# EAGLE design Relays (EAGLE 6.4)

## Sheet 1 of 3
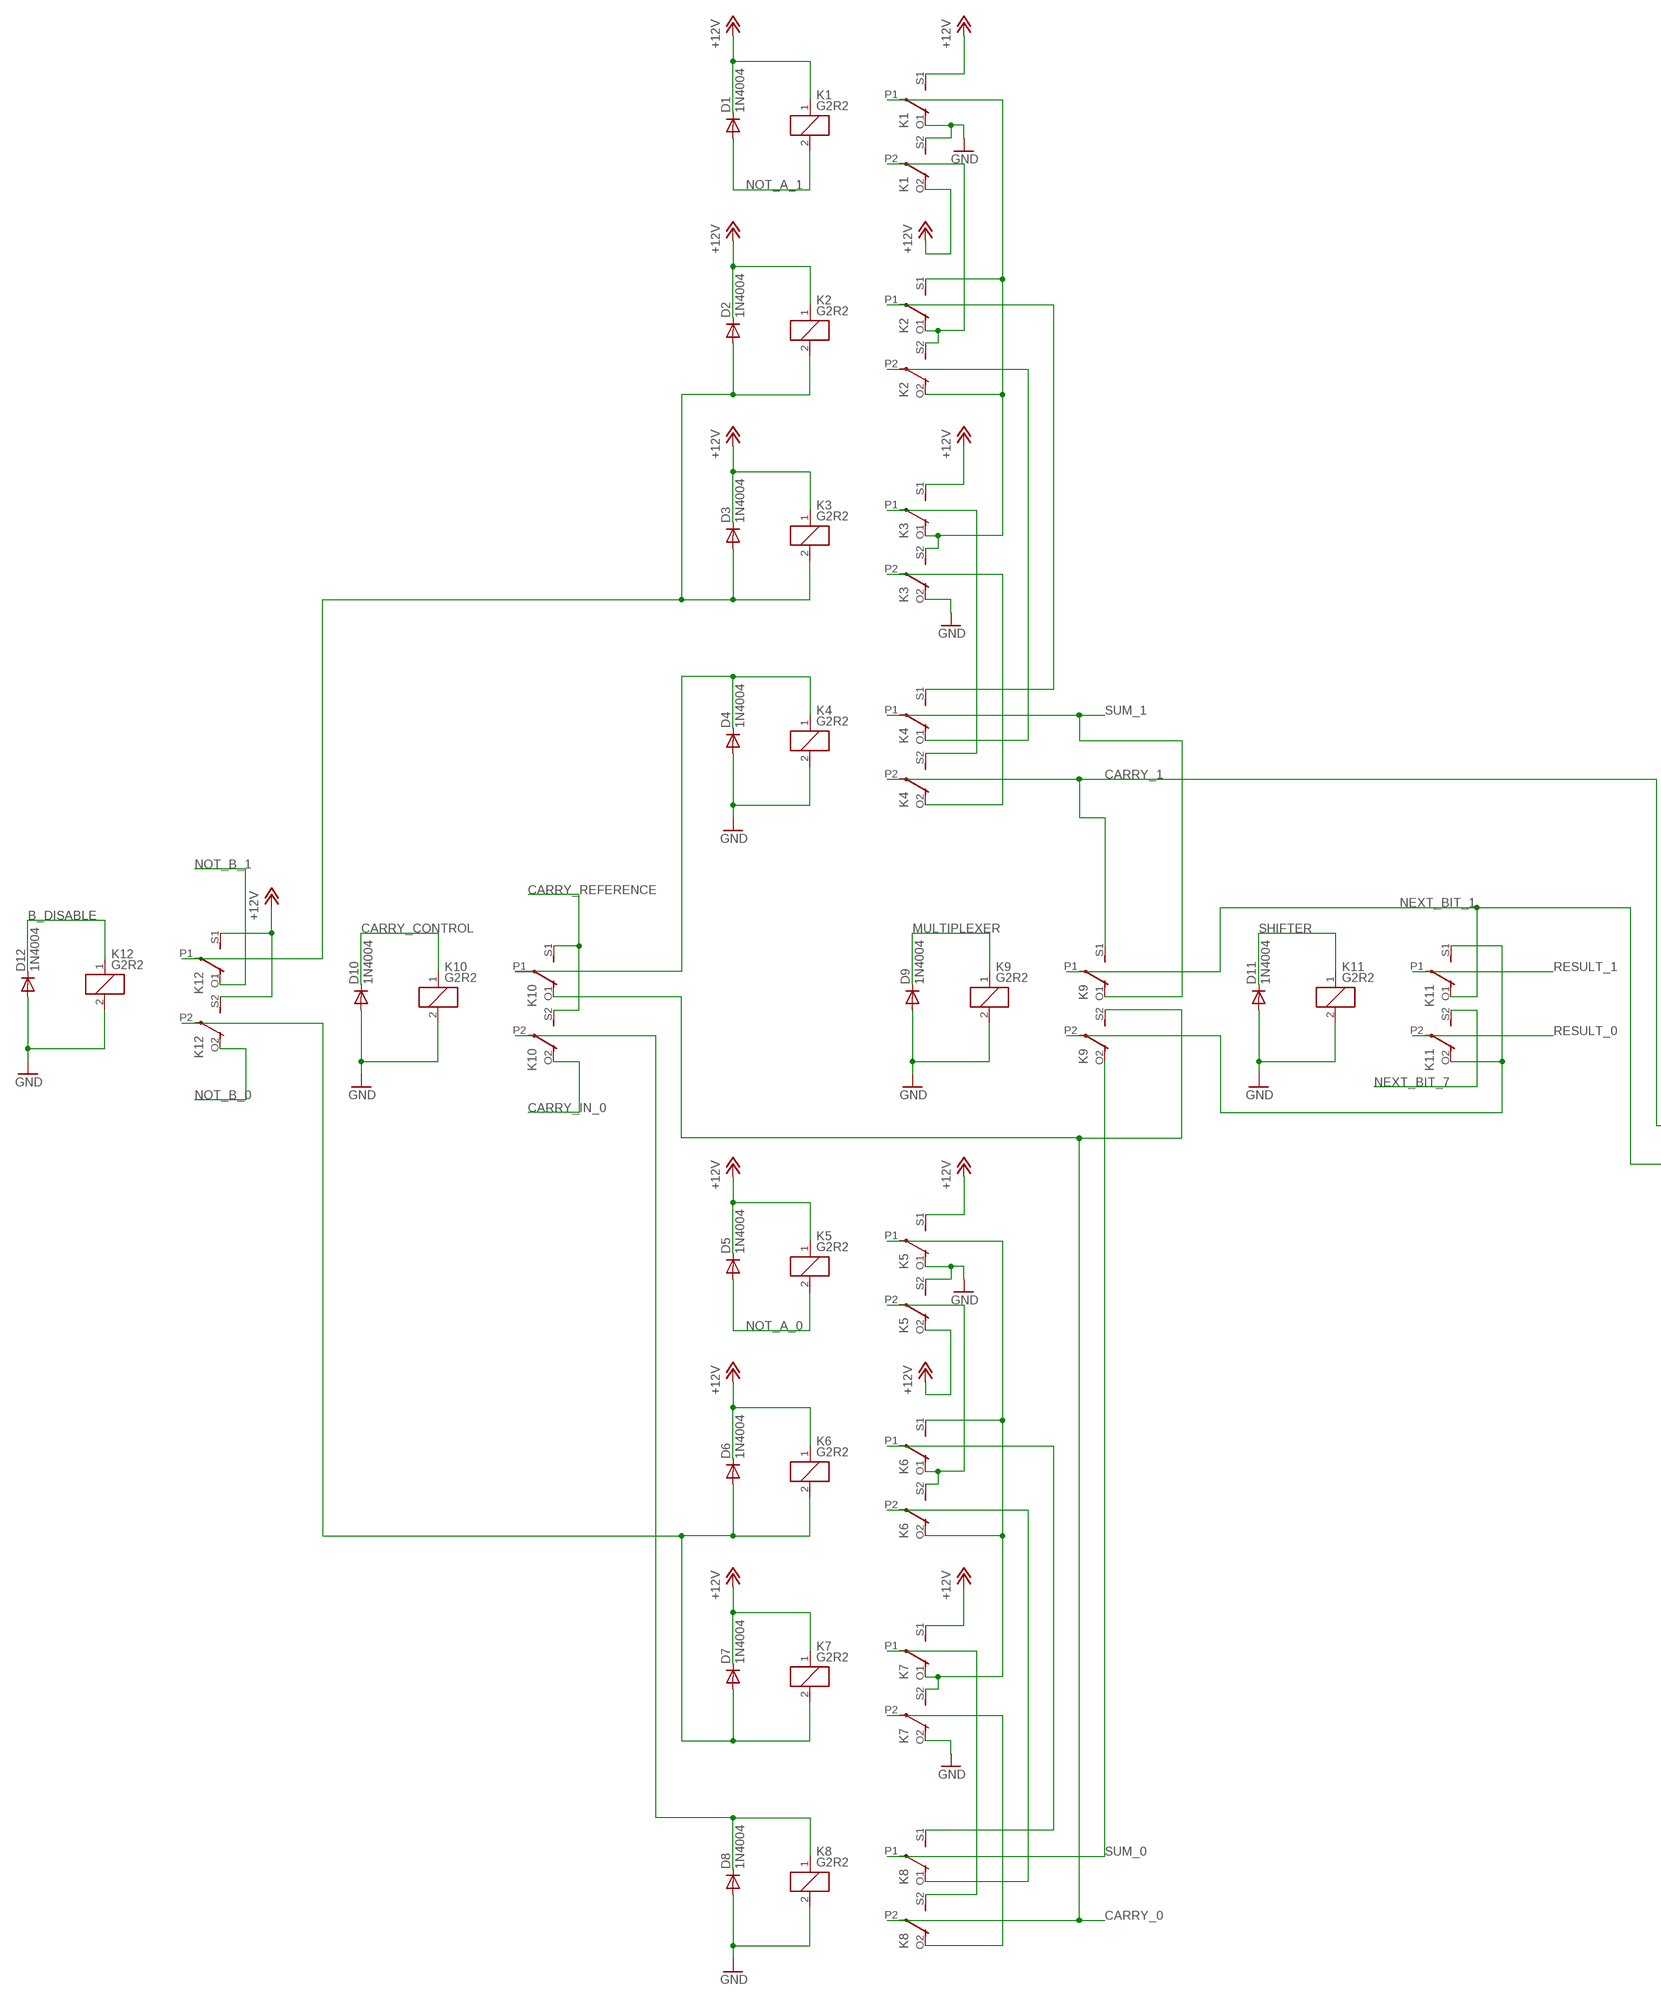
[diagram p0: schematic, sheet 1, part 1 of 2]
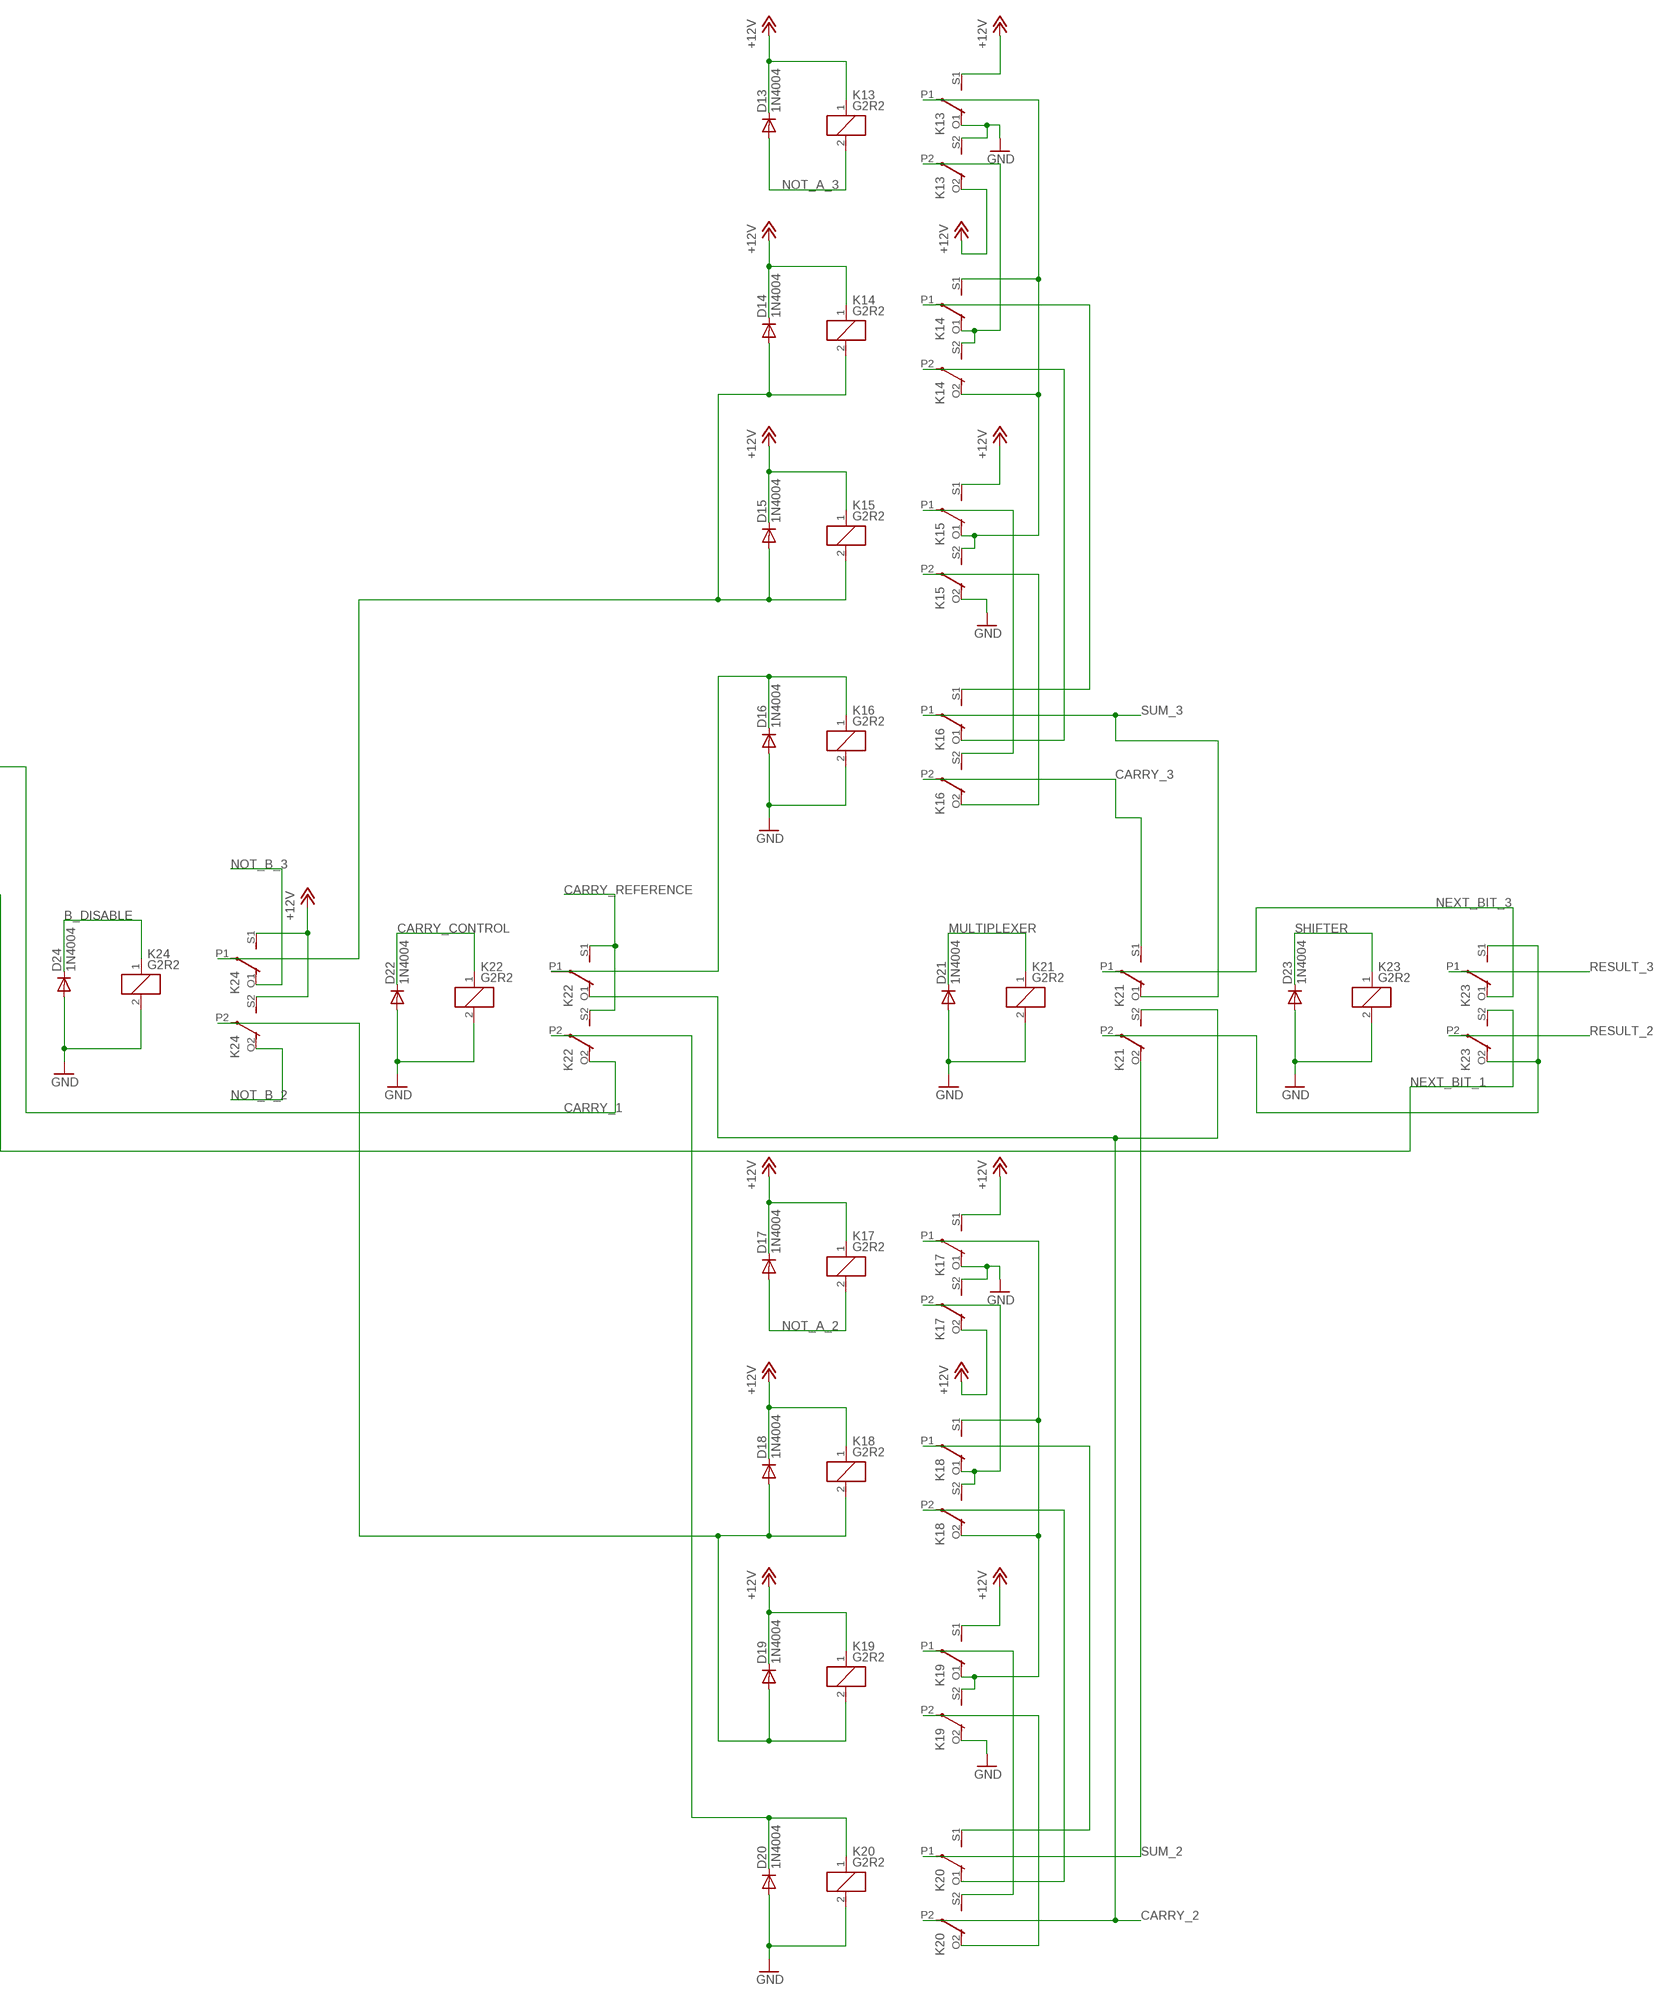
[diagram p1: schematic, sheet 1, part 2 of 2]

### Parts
D1  1N4004  [DO41-10]
D2  1N4004  [DO41-10]
D3  1N4004  [DO41-10]
D4  1N4004  [DO41-10]
D5  1N4004  [DO41-10]
D6  1N4004  [DO41-10]
D7  1N4004  [DO41-10]
D8  1N4004  [DO41-10]
D9  1N4004  [DO41-10]
D10  1N4004  [DO41-10]
D11  1N4004  [DO41-10]
D12  1N4004  [DO41-10]
D13  1N4004  [DO41-10]
D14  1N4004  [DO41-10]
D15  1N4004  [DO41-10]
D16  1N4004  [DO41-10]
D17  1N4004  [DO41-10]
D18  1N4004  [DO41-10]
D19  1N4004  [DO41-10]
D20  1N4004  [DO41-10]
D21  1N4004  [DO41-10]
D22  1N4004  [DO41-10]
D23  1N4004  [DO41-10]
D24  1N4004  [DO41-10]
K1  G2R2  [G2R2]
K2  G2R2  [G2R2]
K3  G2R2  [G2R2]
K4  G2R2  [G2R2]
K5  G2R2  [G2R2]
K6  G2R2  [G2R2]
K7  G2R2  [G2R2]
K8  G2R2  [G2R2]
K9  G2R2  [G2R2]
K10  G2R2  [G2R2]
K11  G2R2  [G2R2]
K12  G2R2  [G2R2]
K13  G2R2  [G2R2]
K14  G2R2  [G2R2]
K15  G2R2  [G2R2]
K16  G2R2  [G2R2]
K17  G2R2  [G2R2]
K18  G2R2  [G2R2]
K19  G2R2  [G2R2]
K20  G2R2  [G2R2]
K21  G2R2  [G2R2]
K22  G2R2  [G2R2]
K23  G2R2  [G2R2]
K24  G2R2  [G2R2]

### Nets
+12V [12V_Power]: D1.C D2.C D3.C D5.C D6.C D7.C D13.C D14.C D15.C D17.C D18.C D19.C K1.1 K1.O2(3:O) K1.S1(2:S) K2.1 K3.1 K3.S1(2:S) K5.1 K5.O2(3:O) K5.S1(2:S) K6.1 K7.1 K7.S1(2:S) K12.S1(2:S) K12.S2(3:S) K13.1 K13.O2(3:O) K13.S1(2:S) K14.1 K15.1 K15.S1(2:S) K17.1 K17.O2(3:O) K17.S1(2:S) K18.1 K19.1 K19.S1(2:S) K24.S1(2:S) K24.S2(3:S) ; also sheet 2,3
B_DISABLE [Relay_Interconnects]: D12.C D24.C K12.1 K24.1 ; also sheet 2,3
CARRY_0 [Relay_Interconnects]: K8.P2(3:P) K9.S2(3:S) K10.O1(2:O)
CARRY_1 [Relay_Interconnects]: K4.P2(3:P) K9.S1(2:S) K22.O2(3:O)
CARRY_2 [Relay_Interconnects]: K20.P2(3:P) K21.S2(3:S) K22.O1(2:O)
CARRY_3: K16.P2(3:P) K21.S1(2:S) ; also sheet 3
CARRY_CONTROL [Relay_Interconnects]: D10.C D22.C K10.1 K22.1 ; also sheet 2,3
CARRY_IN_0 [Relay_Interconnects]: K10.O2(3:O) ; also sheet 2
CARRY_REFERENCE [Relay_Interconnects]: K10.S1(2:S) K10.S2(3:S) K22.S1(2:S) K22.S2(3:S) ; also sheet 2,3
GND [Ground]: D4.A D8.A D9.A D10.A D11.A D12.A D16.A D20.A D21.A D22.A D23.A D24.A K1.O1(2:O) K1.S2(3:S) K3.O2(3:O) K4.2 K5.O1(2:O) K5.S2(3:S) K7.O2(3:O) K8.2 K9.2 K10.2 K11.2 K12.2 K13.O1(2:O) K13.S2(3:S) K15.O2(3:O) K16.2 K17.O1(2:O) K17.S2(3:S) K19.O2(3:O) K20.2 K21.2 K22.2 K23.2 K24.2 ; also sheet 2,3
MULTIPLEXER [Relay_Interconnects]: D9.C D21.C K9.1 K21.1 ; also sheet 2,3
N$1 [Relay_Interconnects]: D2.A D3.A K2.2 K3.2 K12.P1(2:P)
N$3 [Relay_Interconnects]: K9.P2(3:P) K11.O2(3:O) K11.S1(2:S)
N$5 [Relay_Interconnects]: D16.C K16.1 K22.P1(2:P)
N$6: K13.P2(3:P) K14.O1(2:O) K14.S2(3:S)
N$7 [Relay_Interconnects]: D4.C K4.1 K10.P1(2:P)
N$8 [Relay_Interconnects]: D8.C K8.1 K10.P2(3:P)
N$9: K2.P1(2:P) K4.S1(2:S)
N$10: K1.P2(3:P) K2.O1(2:O) K2.S2(3:S)
N$11: K5.P2(3:P) K6.O1(2:O) K6.S2(3:S)
N$12: K1.P1(2:P) K2.O2(3:O) K2.S1(2:S) K3.O1(2:O) K3.S2(3:S)
N$13: K5.P1(2:P) K6.O2(3:O) K6.S1(2:S) K7.O1(2:O) K7.S2(3:S)
N$14: K7.P2(3:P) K8.O2(3:O)
N$15: K3.P2(3:P) K4.O2(3:O)
N$16: K3.P1(2:P) K4.S2(3:S)
N$17: K2.P2(3:P) K4.O1(2:O)
N$18: K7.P1(2:P) K8.S2(3:S)
N$19: K6.P2(3:P) K8.O1(2:O)
N$20: K6.P1(2:P) K8.S1(2:S)
N$21: K13.P1(2:P) K14.O2(3:O) K14.S1(2:S) K15.O1(2:O) K15.S2(3:S)
N$22 [Relay_Interconnects]: D6.A D7.A K6.2 K7.2 K12.P2(3:P)
N$23: K15.P2(3:P) K16.O2(3:O)
N$24: K15.P1(2:P) K16.S2(3:S)
N$25: K14.P2(3:P) K16.O1(2:O)
N$26: K14.P1(2:P) K16.S1(2:S)
N$27 [Relay_Interconnects]: D20.C K20.1 K22.P2(3:P)
N$28: K17.P2(3:P) K18.O1(2:O) K18.S2(3:S)
N$29: K17.P1(2:P) K18.O2(3:O) K18.S1(2:S) K19.O1(2:O) K19.S2(3:S)
N$30: K19.P2(3:P) K20.O2(3:O)
N$31: K19.P1(2:P) K20.S2(3:S)
N$32: K18.P2(3:P) K20.O1(2:O)
N$33: K18.P1(2:P) K20.S1(2:S)
N$34 [Relay_Interconnects]: D14.A D15.A K14.2 K15.2 K24.P1(2:P)
N$35 [Relay_Interconnects]: D18.A D19.A K18.2 K19.2 K24.P2(3:P)
N$36 [Relay_Interconnects]: K21.P2(3:P) K23.O2(3:O) K23.S1(2:S)
NEXT_BIT_1 [Relay_Interconnects]: K9.P1(2:P) K11.O1(2:O) K23.S2(3:S)
NEXT_BIT_3 [Relay_Interconnects]: K21.P1(2:P) K23.O1(2:O) ; also sheet 3
NEXT_BIT_7 [Relay_Interconnects]: K11.S2(3:S) ; also sheet 3
NOT_A_0 [Relay_Interconnects]: D5.A K5.2 ; also sheet 3
NOT_A_1 [Relay_Interconnects]: D1.A K1.2 ; also sheet 3
NOT_A_2 [Relay_Interconnects]: D17.A K17.2 ; also sheet 3
NOT_A_3 [Relay_Interconnects]: D13.A K13.2 ; also sheet 3
NOT_B_0 [Relay_Interconnects]: K12.O2(3:O) ; also sheet 3
NOT_B_1 [Relay_Interconnects]: K12.O1(2:O) ; also sheet 3
NOT_B_2 [Relay_Interconnects]: K24.O2(3:O) ; also sheet 3
NOT_B_3 [Relay_Interconnects]: K24.O1(2:O) ; also sheet 3
RESULT_0 [Relay_Interconnects]: K11.P2(3:P) ; also sheet 3
RESULT_1 [Relay_Interconnects]: K11.P1(2:P) ; also sheet 3
RESULT_2 [Relay_Interconnects]: K23.P2(3:P) ; also sheet 3
RESULT_3 [Relay_Interconnects]: K23.P1(2:P) ; also sheet 3
SHIFTER [Relay_Interconnects]: D11.C D23.C K11.1 K23.1 ; also sheet 2,3
SUM_0: K8.P1(2:P) K9.O2(3:O)
SUM_1 [Relay_Interconnects]: K4.P1(2:P) K9.O1(2:O)
SUM_2: K20.P1(2:P) K21.O2(3:O)
SUM_3 [Relay_Interconnects]: K16.P1(2:P) K21.O1(2:O)

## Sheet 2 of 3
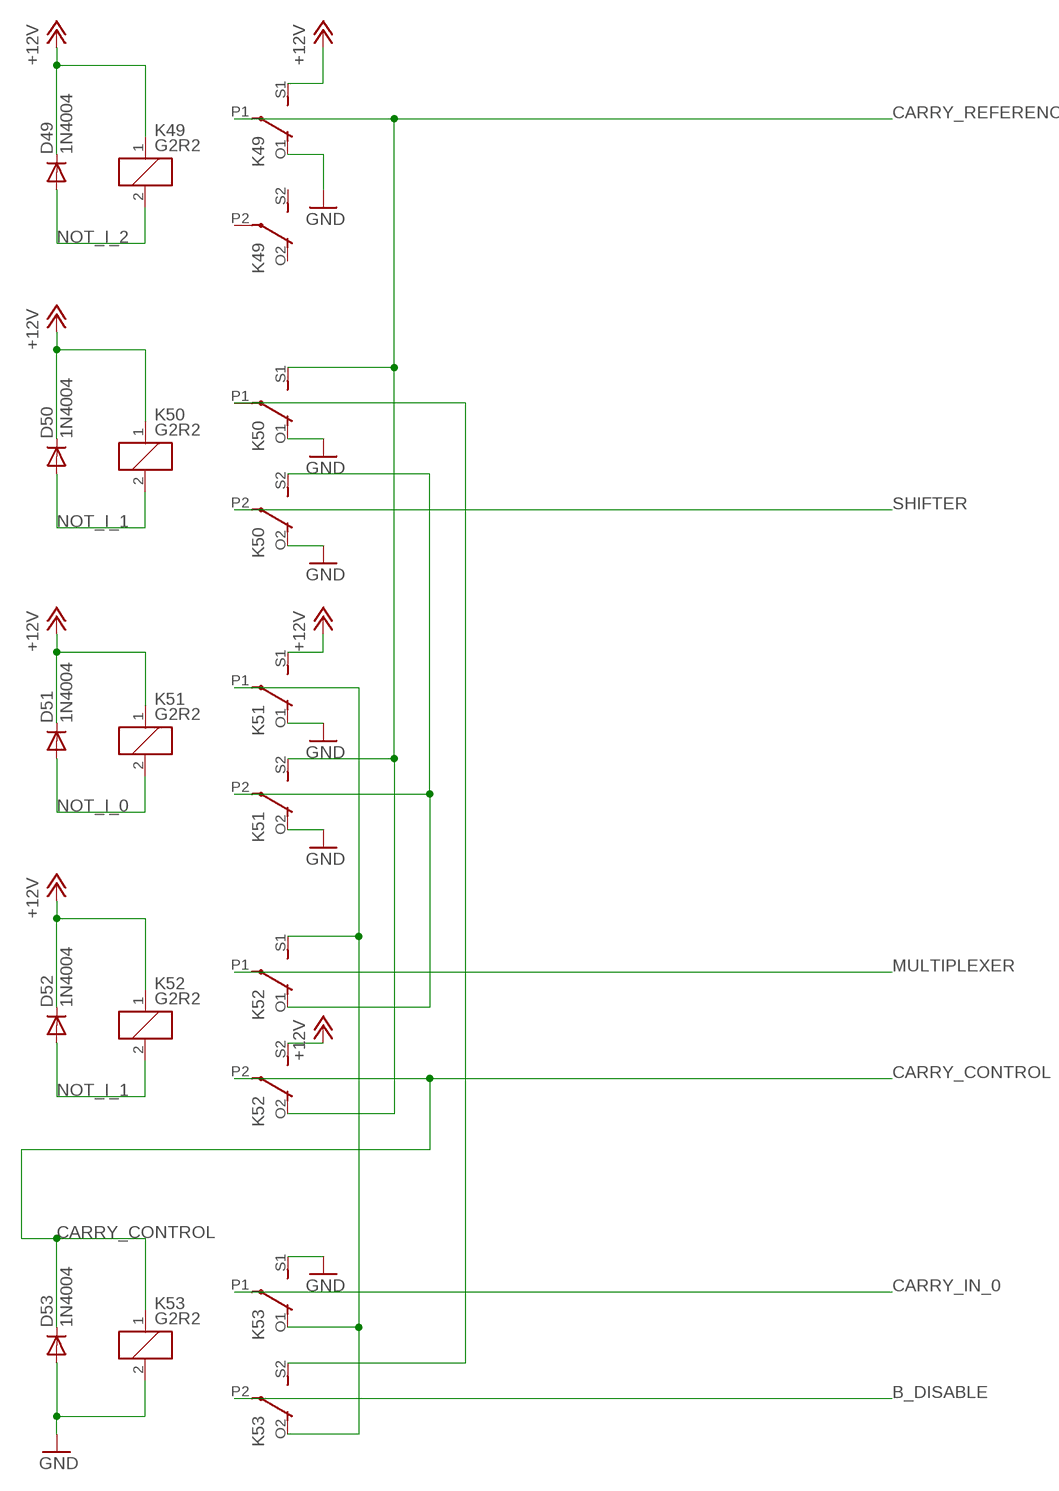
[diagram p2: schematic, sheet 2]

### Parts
D49  1N4004  [DO41-10]
D50  1N4004  [DO41-10]
D51  1N4004  [DO41-10]
D52  1N4004  [DO41-10]
D53  1N4004  [DO41-10]
K49  G2R2  [G2R2]
K50  G2R2  [G2R2]
K51  G2R2  [G2R2]
K52  G2R2  [G2R2]
K53  G2R2  [G2R2]

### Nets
+12V [12V_Power]: D49.C D50.C D51.C D52.C K49.1 K49.S1(2:S) K50.1 K51.1 K51.S1(2:S) K52.1 K52.S2(3:S) ; also sheet 1,3
B_DISABLE [Relay_Interconnects]: K53.P2(3:P) ; also sheet 1,3
CARRY_CONTROL [Relay_Interconnects]: D53.C K52.P2(3:P) K53.1 ; also sheet 1,3
CARRY_IN_0 [Relay_Interconnects]: K53.P1(2:P) ; also sheet 1
CARRY_REFERENCE [Relay_Interconnects]: K49.P1(2:P) K50.S1(2:S) K51.S2(3:S) K52.O2(3:O) ; also sheet 1,3
GND [Ground]: D53.A K49.O1(2:O) K50.O1(2:O) K50.O2(3:O) K51.O1(2:O) K51.O2(3:O) K53.2 K53.S1(2:S) ; also sheet 1,3
MULTIPLEXER [Relay_Interconnects]: K52.P1(2:P) ; also sheet 1,3
N$4: K50.S2(3:S) K51.P2(3:P) K52.O1(2:O)
N$71: K50.P1(2:P) K53.S2(3:S)
N$72: K51.P1(2:P) K52.S1(2:S) K53.O1(2:O) K53.O2(3:O)
NOT_I_0: D51.A K51.2 ; also sheet 3
NOT_I_1: D50.A D52.A K50.2 K52.2 ; also sheet 3
NOT_I_2: D49.A K49.2 ; also sheet 3
SHIFTER [Relay_Interconnects]: K50.P2(3:P) ; also sheet 1,3
Unconnected: K49.O2(3:O) K49.P2(3:P) K49.S2(3:S)

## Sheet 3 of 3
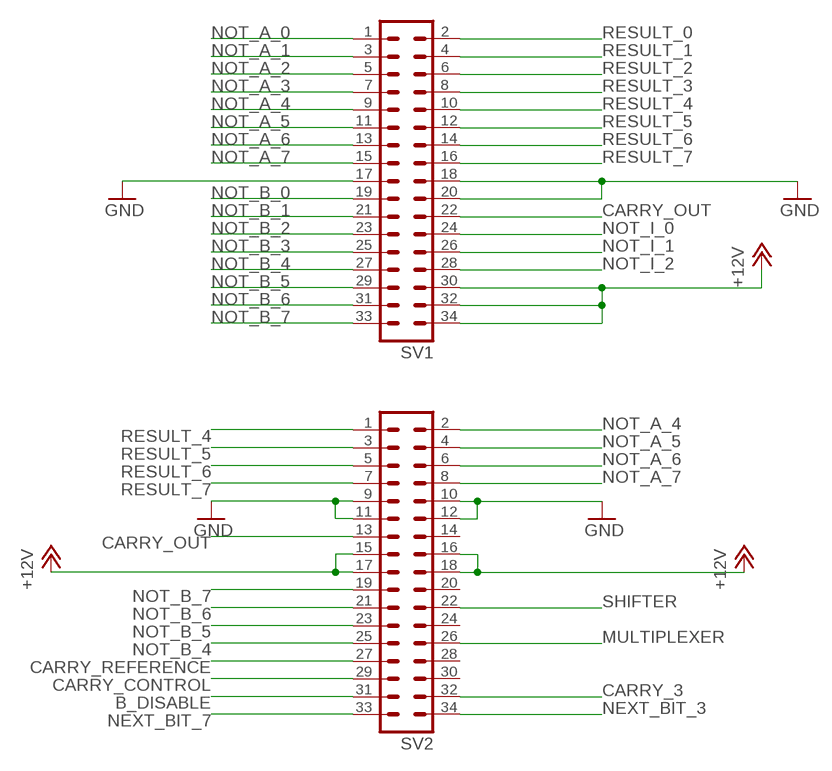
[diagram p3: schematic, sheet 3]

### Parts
SV1  ML34  [ML34]
SV2  ML34  [ML34]

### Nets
+12V [12V_Power]: SV1.30 SV1.32 SV1.34 SV2.15 SV2.16 SV2.17 SV2.18 ; also sheet 1,2
B_DISABLE [Relay_Interconnects]: SV2.31 ; also sheet 1,2
CARRY_3: SV2.32 ; also sheet 1
CARRY_CONTROL [Relay_Interconnects]: SV2.29 ; also sheet 1,2
CARRY_OUT [Relay_Interconnects]: SV1.22 SV2.13
CARRY_REFERENCE [Relay_Interconnects]: SV2.27 ; also sheet 1,2
GND [Ground]: SV1.17 SV1.18 SV1.20 SV2.9 SV2.10 SV2.11 SV2.12 ; also sheet 1,2
MULTIPLEXER [Relay_Interconnects]: SV2.26 ; also sheet 1,2
NEXT_BIT_3 [Relay_Interconnects]: SV2.34 ; also sheet 1
NEXT_BIT_7 [Relay_Interconnects]: SV2.33 ; also sheet 1
NOT_A_0 [Relay_Interconnects]: SV1.1 ; also sheet 1
NOT_A_1 [Relay_Interconnects]: SV1.3 ; also sheet 1
NOT_A_2 [Relay_Interconnects]: SV1.5 ; also sheet 1
NOT_A_3 [Relay_Interconnects]: SV1.7 ; also sheet 1
NOT_A_4 [Relay_Interconnects]: SV1.9 SV2.2
NOT_A_5 [Relay_Interconnects]: SV1.11 SV2.4
NOT_A_6 [Relay_Interconnects]: SV1.13 SV2.6
NOT_A_7 [Relay_Interconnects]: SV1.15 SV2.8
NOT_B_0 [Relay_Interconnects]: SV1.19 ; also sheet 1
NOT_B_1 [Relay_Interconnects]: SV1.21 ; also sheet 1
NOT_B_2 [Relay_Interconnects]: SV1.23 ; also sheet 1
NOT_B_3 [Relay_Interconnects]: SV1.25 ; also sheet 1
NOT_B_4 [Relay_Interconnects]: SV1.27 SV2.25
NOT_B_5 [Relay_Interconnects]: SV1.29 SV2.23
NOT_B_6 [Relay_Interconnects]: SV1.31 SV2.21
NOT_B_7 [Relay_Interconnects]: SV1.33 SV2.19
NOT_I_0: SV1.24 ; also sheet 2
NOT_I_1: SV1.26 ; also sheet 2
NOT_I_2: SV1.28 ; also sheet 2
RESULT_0 [Relay_Interconnects]: SV1.2 ; also sheet 1
RESULT_1 [Relay_Interconnects]: SV1.4 ; also sheet 1
RESULT_2 [Relay_Interconnects]: SV1.6 ; also sheet 1
RESULT_3 [Relay_Interconnects]: SV1.8 ; also sheet 1
RESULT_4 [Relay_Interconnects]: SV1.10 SV2.1
RESULT_5 [Relay_Interconnects]: SV1.12 SV2.3
RESULT_6 [Relay_Interconnects]: SV1.14 SV2.5
RESULT_7 [Relay_Interconnects]: SV1.16 SV2.7
SHIFTER [Relay_Interconnects]: SV2.22 ; also sheet 1,2
Unconnected: SV2.14 SV2.20 SV2.24 SV2.28 SV2.30

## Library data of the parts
D1-D24 D49-D53 = diode:1N4004: DIODE
K1-K24 K49-K53 = relay:G2R2: RELAY 2 x switch, Omron; MF: OMRON COMPONENTS USA; MPN: G2R-2-DC6; OC_FARNELL: unknown; OC_NEWARK: 89C5317
SV1 SV2 = con-harting-ml:ML34: HARTING; OC_FARNELL: unknown; OC_NEWARK: unknown

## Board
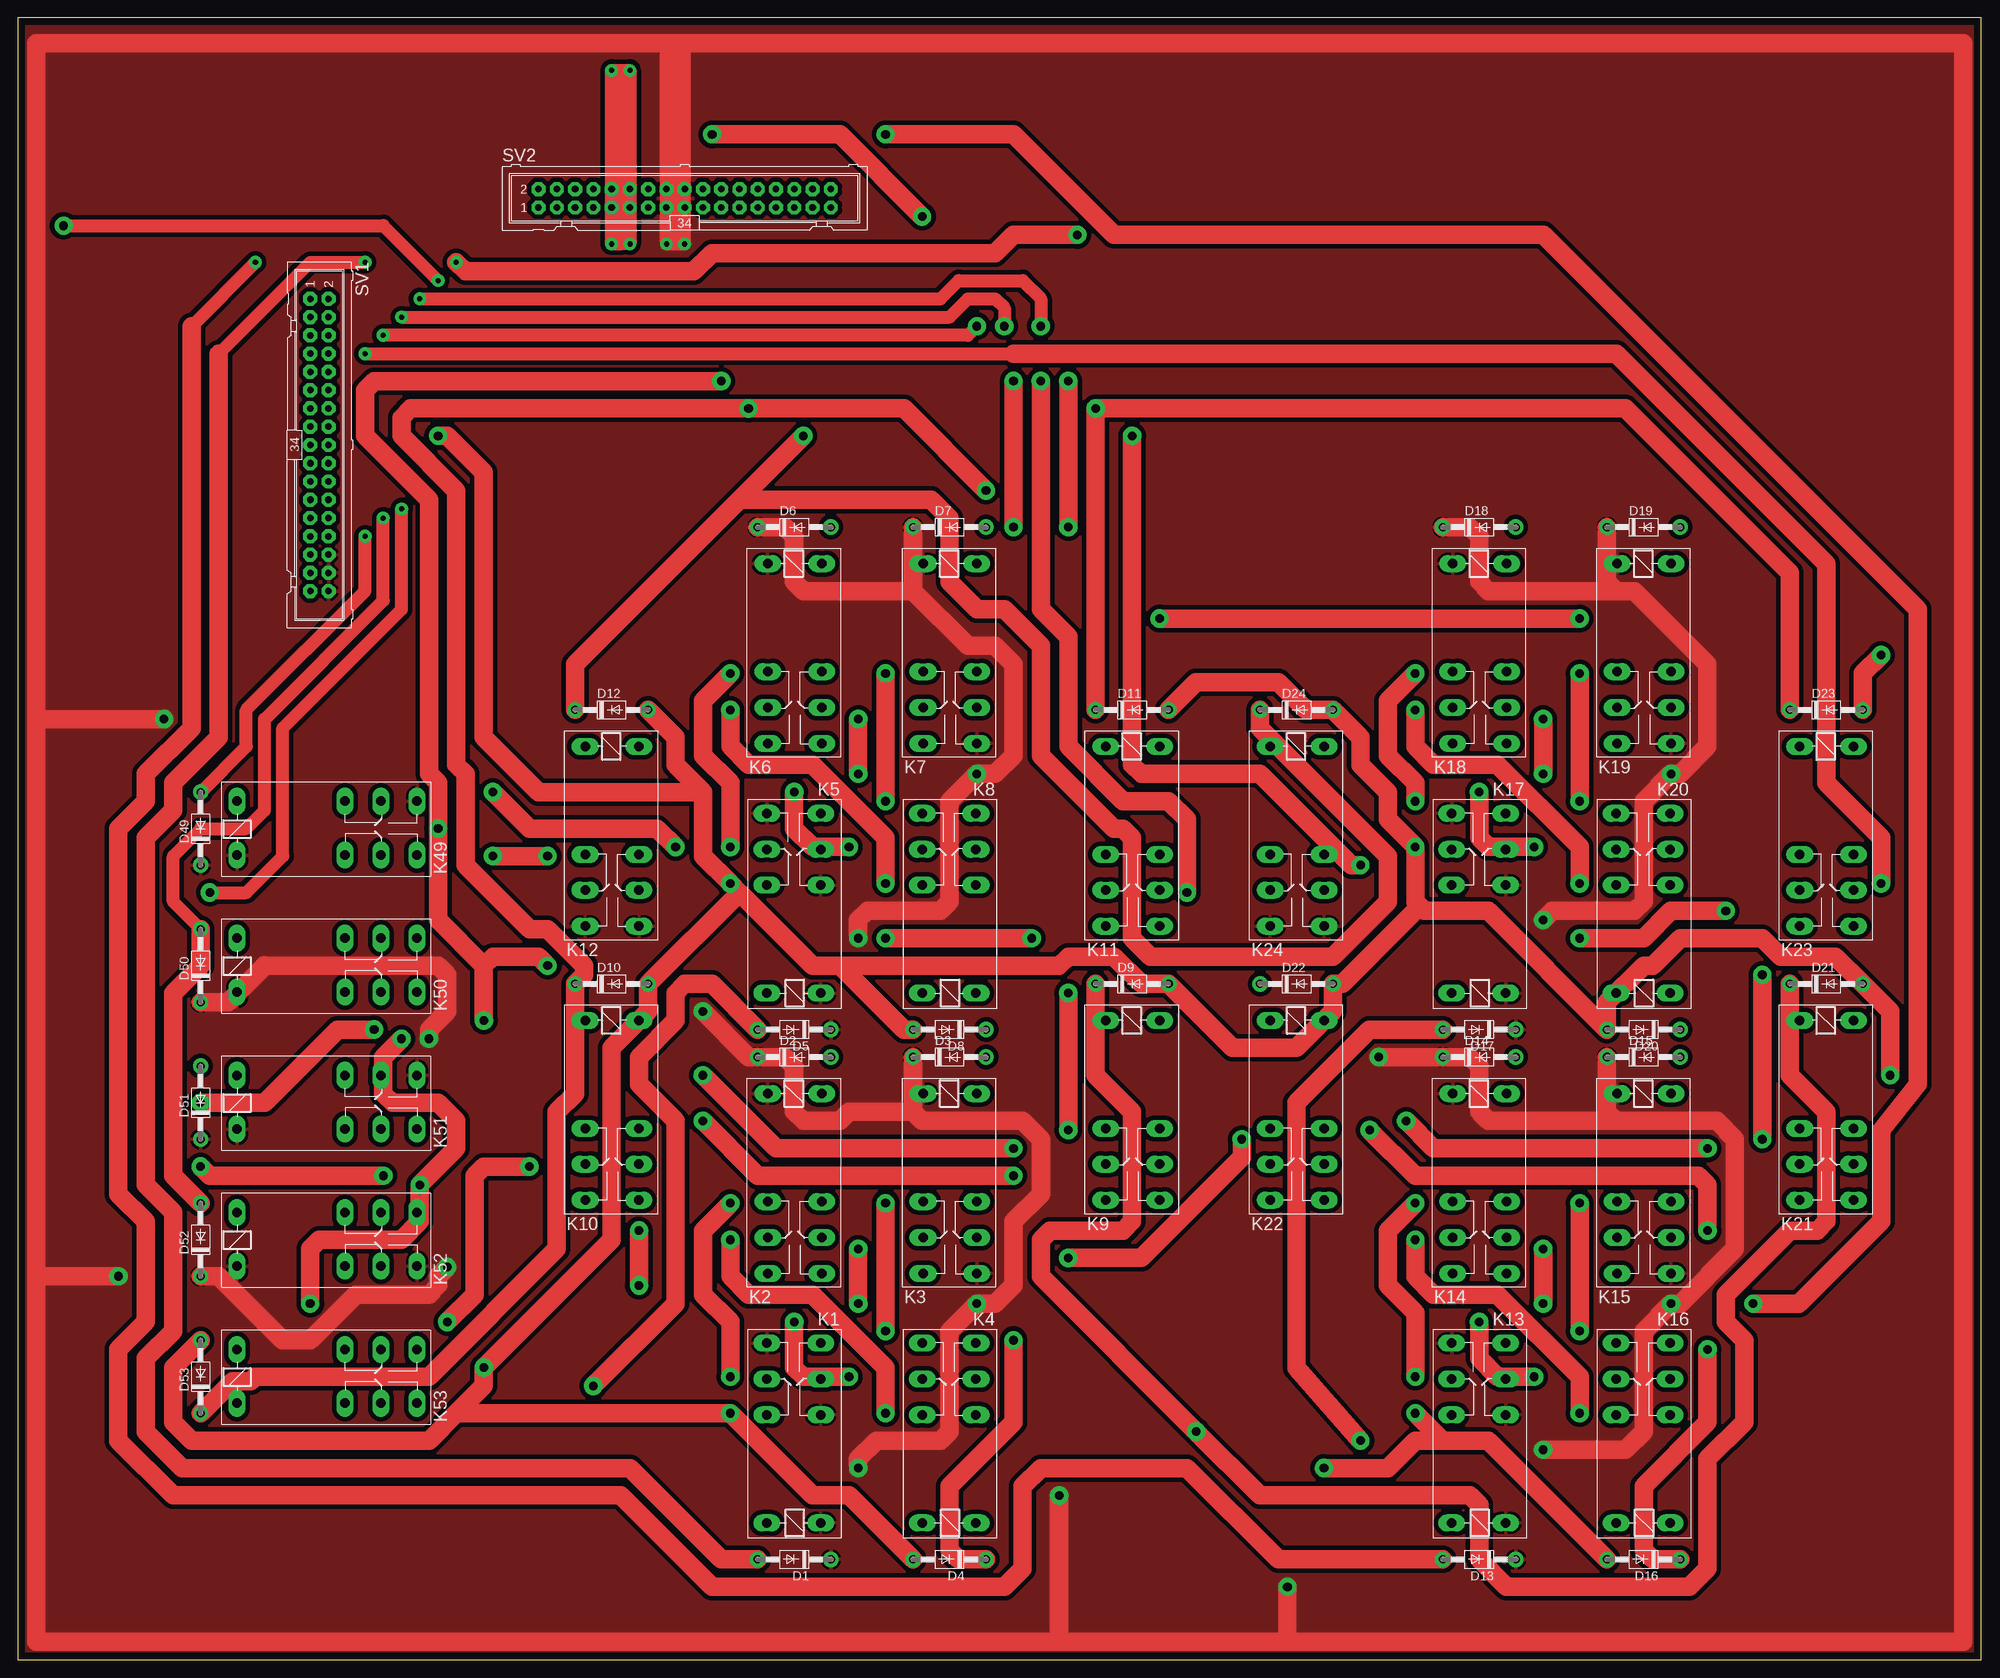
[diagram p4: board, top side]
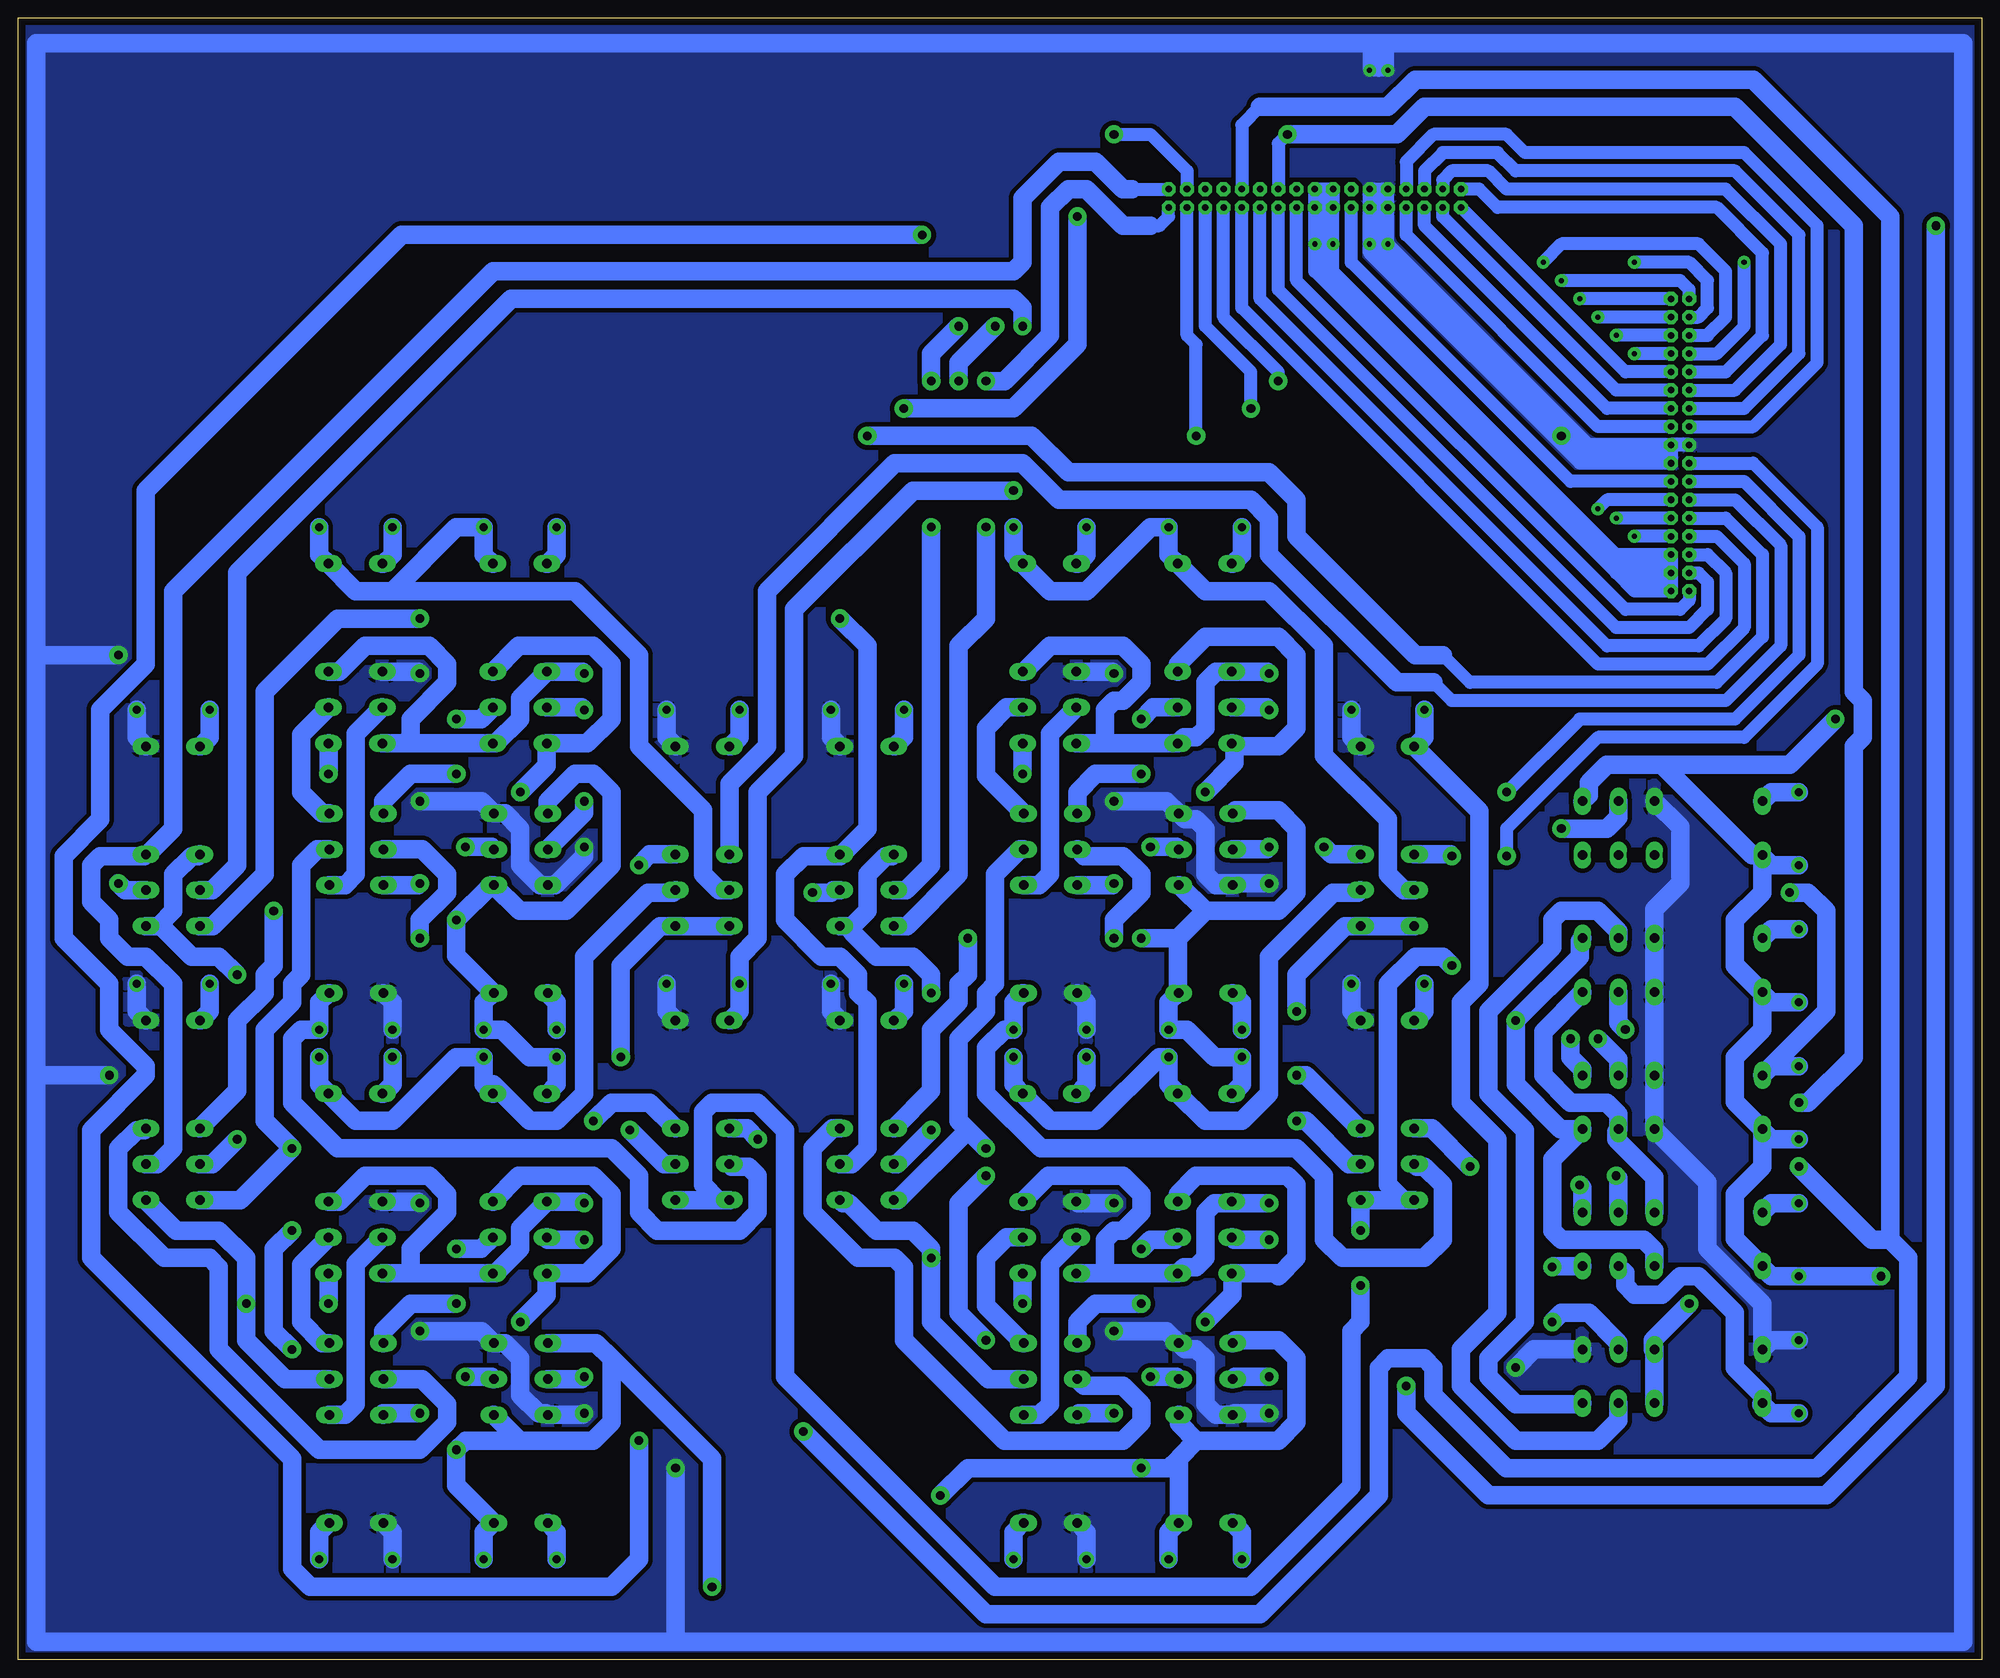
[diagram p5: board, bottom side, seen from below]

Size 273.03 x 228.27 mm. Coordinates in mm from the lower left corner, seen from the top.
Outline: 0,0 273.03,0 273.03,228.27 0,228.27 0,0
Copper layers (1*16): Top 0.035mm / dielectric 1.5mm / Bottom 0.035mm
Design rules "arm-rules-modified": minimum track width 20mil, minimum drill 24mil, track to track 25mil, track to pad 20mil, pad to pad 15mil, via to via 20mil, smd to smd 8mil, copper to edge 40mil, drill to drill 12mil, minimum pad ring 20mil, minimum via ring 20mil, stop-mask expansion 0mil, vias tented up to drill 0mil, thermal gap 15mil

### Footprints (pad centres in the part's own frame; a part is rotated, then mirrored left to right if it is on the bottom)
DO41-10 = drill 1.118: A 5.08,0; C -5.08,0
G2R2 = drill 1.321 long: 1 -2.54,-3.683; 2 -2.54,3.81; O1 12.471,3.81; O2 12.471,-3.683; P1 17.45,3.81; P2 17.45,-3.683; S1 22.454,3.81; S2 22.454,-3.683
ML34 = drill 0.914 octagon: 1 -20.32,-1.27; 2 -20.32,1.27; 3 -17.78,-1.27; 4 -17.78,1.27; 5 -15.24,-1.27; 6 -15.24,1.27; 7 -12.7,-1.27; 8 -12.7,1.27; 9 -10.16,-1.27; 10 -10.16,1.27; 11 -7.62,-1.27; 12 -7.62,1.27; 13 -5.08,-1.27; 14 -5.08,1.27; 15 -2.54,-1.27; 16 -2.54,1.27; 17 0,-1.27; 18 0,1.27; 19 2.54,-1.27; 20 2.54,1.27; 21 5.08,-1.27; 22 5.08,1.27; 23 7.62,-1.27; 24 7.62,1.27; 25 10.16,-1.27; 26 10.16,1.27; 27 12.7,-1.27; 28 12.7,1.27; 29 15.24,-1.27; 30 15.24,1.27; 31 17.78,-1.27; 32 17.78,1.27; 33 20.32,-1.27; 34 20.32,1.27

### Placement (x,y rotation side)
D1  107.95,13.97 180 top
D2  107.95,83.82 0 top
D3  129.54,83.82 0 top
D4  129.54,13.97 180 top
D5  107.95,87.63 180 top
D6  107.95,157.48 0 top
D7  129.54,157.48 0 top
D8  129.54,87.63 180 top
D9  154.94,93.98 0 top
D10  82.55,93.98 0 top
D11  154.94,132.08 0 top
D12  82.55,132.08 0 top
D13  203.2,13.97 180 top
D14  203.2,83.82 0 top
D15  226.06,83.82 0 top
D16  226.06,13.97 180 top
D17  203.2,87.63 180 top
D18  203.2,157.48 0 top
D19  226.06,157.48 0 top
D20  226.06,87.63 180 top
D21  251.46,93.98 0 top
D22  177.8,93.98 0 top
D23  251.46,132.08 0 top
D24  177.8,132.08 0 top
D49  25.4,115.57 90 top
D50  25.4,96.52 90 top
D51  25.4,77.47 90 top
D52  25.4,58.42 90 top
D53  25.4,39.37 90 top
K1  107.95,21.59 90 top
K2  107.95,76.2 270 top
K3  129.54,76.2 270 top
K4  129.54,21.59 90 top
K5  107.95,95.25 90 top
K6  107.95,149.86 270 top
K7  129.54,149.86 270 top
K8  129.54,95.25 90 top
K9  154.94,86.36 270 top
K10  82.55,86.36 270 top
K11  154.94,124.46 270 top
K12  82.55,124.46 270 top
K13  203.2,21.59 90 top
K14  203.2,76.2 270 top
K15  226.06,76.2 270 top
K16  226.06,21.59 90 top
K17  203.2,95.25 90 top
K18  203.2,149.86 270 top
K19  226.06,149.86 270 top
K20  226.06,95.25 90 top
K21  251.46,86.36 270 top
K22  177.8,86.36 270 top
K23  251.46,124.46 270 top
K24  177.8,124.46 270 top
K49  33.02,115.57 0 top
K50  33.02,96.52 0 top
K51  33.02,77.47 0 top
K52  33.02,58.42 0 top
K53  33.02,39.37 0 top
SV1  41.91,168.91 270 top
SV2  92.71,203.2 0 top

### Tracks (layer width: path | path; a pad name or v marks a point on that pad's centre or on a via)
+12V  (via drill 0.7 pad 1.78, 1.2 pad 2.54)
  Top 1.778: 90.17,224.79 v90.17,196.85 v92.71,196.85 | v92.71,196.85 92.71,224.79 | v92.71,196.85 91.44,198.12 91.44,224.79
  Top 2.54: 124.46,148.59 132.08,140.97 135.89,140.97 138.43,138.43 138.43,125.73 135.89,123.19 v133.35,123.19 129.54,119.38 129.54,105.41 128.27,104.14 118.11,104.14 116.84,102.87 v116.84,100.33 | 124.46,148.59 D7.C | v116.84,26.67 116.84,27.94 119.38,30.48 128.27,30.48 129.54,31.75 129.54,45.72 v133.35,49.53 135.89,49.53 138.43,52.07 138.43,60.96 142.24,64.77 142.24,72.39 139.7,74.93 125.73,74.93 124.46,76.2 | 124.46,76.2 D3.C | v212.09,29.21 223.52,29.21 226.06,31.75 226.06,45.72 v229.87,49.53 231.14,49.53 238.76,57.15 238.76,72.39 236.22,74.93 222.25,74.93 | 222.25,74.93 220.98,76.2 D15.C | 222.25,148.59 224.79,148.59 234.95,138.43 234.95,127 231.14,123.19 v229.87,123.19 226.06,119.38 226.06,105.41 224.79,104.14 213.36,104.14 v212.09,102.87 | 222.25,148.59 220.98,149.86 D19.C | 124.46,76.2 115.57,76.2 114.3,74.93 109.22,74.93 107.95,76.2 107.95,82.55 106.68,83.82 D2.C 101.6,83.82 v95.25,90.17 | 124.46,148.59 109.22,148.59 107.95,149.86 107.95,156.21 106.68,157.48 D6.C | 222.25,74.93 204.47,74.93 203.2,76.2 203.2,82.55 201.93,83.82 D14.C v189.23,83.82 | 222.25,148.59 204.47,148.59 203.2,149.86 203.2,156.21 201.93,157.48 D18.C | v57.15,86.36 57.15,87.63 59.69,90.17 59.69,95.25 58.42,96.52 34.29,96.52 34.23,96.58 34.23,96.46 29.21,91.44 D50.C | D52.C 27.94,53.34 36.83,44.45 40.64,44.45 46.99,50.8 57.15,50.8 58.42,52.07 58.42,53.34 v59.69,54.61 | 144.78,2.54 2.54,2.54 2.54,53.34 | 144.78,2.54 176.53,2.54 | 176.53,2.54 270.51,2.54 270.51,224.79 92.71,224.79 91.44,224.79 90.17,224.79 2.54,224.79 2.54,130.81 | 2.54,130.81 2.54,53.34 | v13.97,53.34 2.54,53.34
  Top 2.54: v20.32,130.81 2.54,130.81 | v144.78,22.86 144.78,2.54 | v176.53,10.16 176.53,2.54
  Bottom 1.778: SV2.16 SV2.15 | 92.71,203.2 SV2.18 | SV2.17 91.44,203.2 | SV1.30 50.8,153.67 90.17,193.04 v90.17,196.85 SV2.15 | 43.18,152.4 50.8,152.4 91.44,193.04 91.44,201.93 | SV1.32 49.53,151.13 | 49.53,151.13 50.8,151.13 | 50.8,151.13 92.71,193.04 v92.71,196.85 SV2.17 | 91.44,203.2 SV2.16 | SV2.16 SV2.18 | SV2.18 91.44,203.2 | 91.44,203.2 SV2.15 | SV2.15 91.44,201.93 | 91.44,201.93 SV2.17 | SV2.17 92.71,203.2 | 92.71,203.2 91.44,203.2 | 91.44,203.2 91.44,201.93 | SV1.34 48.26,148.59 50.8,151.13 | 43.18,149.86 48.26,149.86 49.53,151.13
  Bottom 1.93: SV1.30 43.18,152.4 SV1.32 43.18,149.86 SV1.34
  Bottom 2.54: D3.C 124.46,80.01 125.73,78.74 K3.1 | D1.C 113.03,17.78 111.76,19.05 K1.1 111.63,28.07 | 111.76,92.71 113.03,91.44 D5.C 110.49,87.63 106.68,83.82 D2.C 102.87,80.01 104.14,78.74 K2.1 | D7.C 124.46,153.67 125.73,152.4 K7.1 | D13.C 208.28,17.78 207.01,19.05 K13.1 212.09,24.26 v212.09,29.21 210.82,30.48 203.3,30.48 | D15.C 220.98,80.01 222.25,78.74 K15.1 | D18.C 198.12,153.67 199.39,152.4 K18.1 | D19.C 220.98,153.67 222.25,152.4 K19.1 | D49.C 29.21,110.49 30.48,111.76 | D50.C 29.21,91.44 30.48,92.71 | D51.C 29.21,72.39 30.48,73.66 30.48,68.58 34.29,64.77 34.29,58.55 K52.1 30.48,54.61 29.21,53.34 D52.C v13.97,53.34 | K7.S1 v133.35,123.19 | K5.O2 111.53,107.72 107.95,104.14 | 107.95,104.14 97.79,104.14 95.25,106.68 95.25,115.57 97.79,118.11 103.73,118.11 K5.S1 | 111.76,92.71 111.76,100.33 | 111.76,100.33 107.95,104.14 | K6.1 104.14,152.4 102.87,153.67 D6.C | v116.84,100.33 111.76,100.33 | K3.S1 v133.35,49.53 | K1.S1 103.73,44.45 97.79,44.45 95.25,41.91 95.25,33.02 97.79,30.48 109.22,30.48 | 109.22,30.48 111.63,32.89 K1.O2 | 109.22,30.48 111.63,28.07 | 111.63,28.07 113.03,26.67 v116.84,26.67 140.97,26.67 v144.78,22.86 | K13.O2 203.3,30.48 | 203.3,30.48 193.04,30.48 190.5,33.02 190.5,41.91 | 190.5,41.91 192.63,44.04 K13.S1 | K15.S1 v229.87,49.53 | K19.S1 v229.87,123.19 | K12.S2 K12.S1 88.49,102.01 95.25,95.25 v95.25,90.17 | K24.S2 K24.S1 183.74,102.01 189.23,96.52 v189.23,83.82 | 30.48,111.76 30.48,106.68 34.29,102.87 34.29,96.65 | 34.29,96.65 K50.1 | 30.48,92.71 30.48,87.63 34.29,83.82 34.29,77.6 K51.1 | 44.45,124.46 31.88,111.89 K49.1 30.48,111.76 | 44.45,124.46 52.07,124.46 54.61,121.92 54.61,120.24 K49.S1
  Bottom 2.54: K51.S1 55.47,82.14 57.15,83.82 v57.15,86.36 | K52.S2 59.56,54.74 v59.69,54.61 | v176.53,10.16 176.53,27.94 190.5,41.91 | 199.8,117.7 K17.S1 199.39,119.38 195.58,123.19 193.04,123.19 190.5,120.65 190.5,110.49 196.85,104.14 203.3,104.14 K17.O2 207.24,107.72 v212.09,102.87 212.09,97.92 K17.1 207.01,92.71 208.28,91.44 D17.C 205.74,87.63 201.93,83.82 D14.C 198.12,80.01 199.39,78.74 K14.1 | 34.29,96.65 34.29,96.52 30.48,92.71 | 111.76,92.71 K5.1 | 44.45,124.46 26.67,124.46 v20.32,130.81
  pour Top: 0,228.6 273.05,228.6 273.05,0 0,0
B_DISABLE  (via drill 1.2 pad 2.54)
  Top 2.54: D12.C 77.47,138.43 100.33,161.29 | 100.33,161.29 127,161.29 129.54,158.75 129.54,149.86 133.35,146.05 137.16,146.05 142.24,140.97 142.24,125.73 152.4,115.57 153.67,115.57 154.94,114.3 154.94,100.33 157.48,97.79 182.88,97.79 190.5,105.41 190.5,111.76 172.72,129.54 D24.C | 100.33,161.29 v109.22,170.18
  Bottom 1.778: v109.22,170.18 109.22,182.88 110.49,184.15 SV2.31
  Bottom 2.54: D12.C 77.47,128.27 78.74,127 K12.1 69.85,117.98 69.85,93.98 72.39,91.44 72.39,77.47 67.31,72.39 67.31,48.26 72.39,43.18 72.39,38.1 64.77,30.48 53.34,30.48 50.47,33.35 K53.P2 | D24.C 172.72,128.27 173.99,127 K24.1
CARRY_0  (via drill 1.2 pad 2.54)
  Top 2.54: v138.43,71.12 105.41,71.12 v95.25,81.28
  Bottom 2.54: K8.P2 133.68,112.7 137.16,109.22 137.16,93.98 138.43,92.71 138.43,90.17 142.24,86.36 142.24,74.93 140.97,73.66 | 140.97,73.66 v138.43,71.12 | K9.S2 150.72,63.91 140.97,73.66 | K10.O1 86.59,73.89 93.98,81.28 v95.25,81.28
CARRY_1  (via drill 1.2 pad 2.54)
  Top 2.54: v146.05,55.88 156.21,55.88 170.18,69.85 v170.18,72.39
  Bottom 2.54: K9.S1 158.34,63.5 157.48,63.5 153.67,59.69 148.59,59.69 146.05,57.15 v146.05,55.88 146.05,46.99 138.1,39.04 K4.P2 | K22.O2 171.68,73.89 v170.18,72.39
CARRY_2  (via drill 1.2 pad 2.54)
  Top 2.54: v193.04,74.93 196.85,71.12 v234.95,71.12
  Bottom 2.54: K22.O1 185.19,77.47 190.5,77.47 v193.04,74.93 | K20.P2 231.47,112.7 233.68,110.49 233.68,95.25 234.95,93.98 234.95,91.44 238.76,87.63 238.76,74.93 v234.95,71.12 242.16,63.91 K21.S2
CARRY_3  (via drill 1.2 pad 2.54)
  Top 2.54: v241.3,49.53 247.65,49.53 259.08,60.96 259.08,73.66 264.16,80.01 264.16,146.05 212.09,198.12 152.4,198.12 138.43,212.09 v120.65,212.09
  Bottom 1.778: v120.65,212.09 115.57,212.09 110.49,207.01 SV2.32
  Bottom 2.54: K16.P2 235.89,39.04 241.3,44.45 v241.3,49.53 241.3,55.88 245.11,59.69 251.05,59.69 K21.S1
CARRY_CONTROL  (via drill 1.2 pad 2.54)
  Top 2.54: D53.C 29.84,38.73 32.38,38.73 33.02,39.37 57.15,39.37 74.93,57.15 74.93,76.2 77.47,78.74 D10.C 78.74,95.25 78.74,96.52 73.66,101.6 71.12,101.6 62.23,110.49 62.23,123.19 60.96,124.46 60.96,162.56 53.34,170.18 53.34,172.72 54.61,173.99 v101.6,173.99 123.19,173.99 v134.62,162.56
  Bottom 1.778: v101.6,173.99 101.6,179.07 107.95,185.42 SV2.29
  Bottom 2.54: D10.C 77.47,90.17 78.74,88.9 K10.1 | D53.C 29.21,34.29 30.48,35.56 K53.1 | 30.61,35.56 K53.1 | K53.1 30.48,36.83 34.29,40.64 34.29,48.26 39.37,53.34 41.91,53.34 44.45,50.8 48.26,50.8 49.53,52.07 49.53,53.8 K52.P2 | v134.62,162.56 148.59,162.56 165.1,146.05 165.1,125.73 170.18,120.65 170.18,100.33 172.72,97.79 D22.C 172.72,90.17 173.99,88.9 K22.1
CARRY_IN_0  (via drill 1.2 pad 2.54)
  Top 2.54: v59.69,46.99 63.5,50.8 63.5,67.31 64.77,68.58 v71.12,68.58
  Bottom 2.54: K53.P1 50.47,44.12 54.61,48.26 58.42,48.26 v59.69,46.99 | K10.O2 76.43,73.89 v71.12,68.58
CARRY_OUT
  Bottom 1.778: SV1.22 57.15,163.83 87.63,194.31 SV2.13
CARRY_REFERENCE  (via drill 1.2 pad 2.54)
  Top 2.54: v64.77,88.9 64.77,96.52 | 64.77,96.52 58.42,102.87 v58.42,115.57 58.42,121.92 57.15,123.19 57.15,161.29 48.26,170.18 48.26,176.53 49.53,177.8 v97.79,177.8 | 64.77,96.52 66.04,97.79 72.39,97.79 v73.66,96.52 | v86.36,52.07 v86.36,59.69
  Bottom 1.778: v97.79,177.8 97.79,179.07 105.41,186.69 SV2.27
  Bottom 2.54: K22.S1 K22.S2 175.67,63.91 177.8,66.04 177.8,76.2 176.53,77.47 170.18,77.47 166.37,73.66 166.37,39.37 137.16,10.16 101.6,10.16 87.63,24.13 87.63,45.72 86.36,46.99 v86.36,52.07 | K49.P1 50.47,117.17 52.07,115.57 v58.42,115.57 | K50.S1 55.88,99.92 55.88,97.79 v64.77,88.9 64.77,80.01 58.55,73.79 K51.S2 59.69,69.57 59.69,59.69 58.42,58.42 46.99,58.42 45.49,56.92 K52.O2 | v86.36,59.69 K10.S1 K10.S2 80.42,63.91 82.55,66.04 82.55,93.98 78.74,97.79 74.93,97.79 v73.66,96.52
GND  (via drill 0.7 pad 1.78, 1.2 pad 2.54)
  Top 1.778: v82.55,196.85 v82.55,220.98 v85.09,220.98 v85.09,196.85 83.82,196.85 | 83.82,196.85 83.82,198.12 | 83.82,220.98 83.82,198.12 | 83.82,198.12 v82.55,196.85 | v82.55,196.85 83.82,196.85
  Top 2.54: v120.65,137.16 v120.65,119.38 | 100.33,106.68 v99.06,107.95 95.25,111.76 95.25,120.65 | 100.33,106.68 110.49,96.52 114.3,96.52 | 114.3,96.52 123.19,87.63 D8.A | D4.A 115.57,22.86 110.49,22.86 v99.06,34.29 60.96,34.29 | v120.65,63.5 v120.65,45.72 | v217.17,45.72 v217.17,63.5 | v217.17,119.38 v217.17,137.16 | D16.A 204.47,30.48 198.12,30.48 | 198.12,30.48 v194.31,34.29 | 194.94,104.78 194.31,105.41 v194.31,113.03 190.5,116.84 190.5,120.65 186.69,124.46 186.69,128.27 D24.A 179.07,132.08 175.26,135.89 163.83,135.89 D11.A | 194.94,104.78 195.58,104.14 204.47,104.14 D20.A 220.98,91.44 226.06,96.52 227.33,96.52 231.14,100.33 242.57,100.33 245.11,97.79 252.73,97.79 D21.A 260.35,90.17 v260.35,81.28 | 100.33,106.68 D10.A 87.63,90.17 82.55,85.09 82.55,58.42 v64.77,40.64 64.77,38.1 60.96,34.29 | 194.94,104.78 184.15,93.98 D22.A 182.88,90.17 177.8,85.09 168.91,85.09 D9.A 156.21,93.98 152.4,97.79 146.05,97.79 144.78,96.52 114.3,96.52 | 95.25,120.65 91.44,124.46 91.44,128.27 D12.A | D53.A 21.59,40.64 21.59,33.02 24.13,30.48 57.15,30.48 60.96,34.29 | 198.12,30.48 194.31,30.48 190.5,26.67 v181.61,26.67 | 95.25,120.65 72.39,120.65 64.77,128.27 64.77,165.1 59.69,170.18 v58.42,170.18 | D23.A 256.54,137.16 v259.08,139.7
  Bottom 1.778: SV2.9 SV2.11 | SV2.11 SV2.12 83.82,204.47 | SV2.9 SV2.10 83.82,204.47 | SV1.18 54.61,168.91 v82.55,196.85 SV2.9 | SV1.20 55.88,166.37 | SV2.11 v85.09,196.85 85.09,195.58 55.88,166.37 | 43.18,167.64 48.26,167.64 | 83.82,196.85 83.82,203.2 83.82,204.47 | 54.61,167.64 55.88,166.37 | 82.55,224.79 v82.55,220.98 83.82,220.98 | 83.82,220.98 v85.09,220.98 | 83.82,222.25 83.82,224.79 85.09,223.52 | 83.82,222.25 83.82,220.98 | v85.09,220.98 85.09,223.52 | 85.09,224.79 85.09,223.52 | 85.09,223.52 83.82,222.25 | 83.82,222.25 v85.09,220.98 | 85.09,223.52 v85.09,220.98
  Bottom 1.93: SV1.17 SV1.18 43.18,167.64 SV1.20
  Bottom 2.54: D12.A 87.63,128.27 K12.2 | D10.A 87.63,90.17 K10.2 | D9.A 160.02,90.17 K9.2 | D4.A 124.46,17.78 K4.2 | D8.A 124.46,91.44 K8.2 | D11.A 160.02,128.27 K11.2 | D24.A 182.88,128.27 K24.2 | D22.A 182.88,90.17 K22.2 | D21.A 256.54,90.17 K21.2 | D23.A 256.54,128.27 K23.2 | D16.A 220.98,17.78 K16.2 | D20.A 220.98,91.44 K20.2 | D53.A 29.21,44.45 K53.2 30.48,49.53 38.1,57.15 38.1,66.4 K51.O2 K51.O1 K50.O2 K50.O1 45.49,104.37 41.91,107.95 41.91,115.8 K49.O1 | K7.O2 120.88,137.39 v120.65,137.16 | K5.O1 106.45,107.72 106.68,107.95 | v120.65,119.38 113.31,119.38 K5.S2 110.77,116.84 109.22,116.84 107.95,115.57 107.95,109.22 106.68,107.95 | 106.68,107.95 v99.06,107.95 | K3.O2 125.63,63.5 v120.65,63.5 | v120.65,45.72 113.31,45.72 K1.S2 110.77,43.18 109.22,43.18 107.95,41.91 107.95,35.56 106.45,34.06 K1.O1 103.91,34.29 v99.06,34.29 | K15.O2 217.4,63.73 v217.17,63.5 | v194.31,34.29 194.54,34.06 K13.O1 199.62,34.29 200.66,34.29 203.2,36.83 203.2,41.91 205.33,44.04 K13.S2 208.56,45.72 v217.17,45.72 | K19.O2 217.4,137.39 v217.17,137.16 | v217.17,119.38 208.56,119.38 K17.S2 205.33,117.7 203.2,115.57 203.2,110.49 200.43,107.72 K17.O1 198.35,107.72 194.31,111.76 v194.31,113.03 | K53.S1 62.23,43.18 v64.77,40.64 | 181.61,2.54 2.54,2.54 2.54,224.79 82.55,224.79 83.82,224.79 85.09,224.79 270.51,224.79 270.51,139.7 | 181.61,2.54 270.51,2.54 270.51,81.28 | 270.51,81.28 270.51,139.7 | v260.35,81.28 270.51,81.28 | v259.08,139.7 270.51,139.7 | v181.61,26.67 181.61,2.54 | 48.26,167.64 54.61,167.64 55.88,167.64 v58.42,170.18 83.82,195.58 83.82,203.2
  pour Bottom: 0,228.6 273.05,228.6 273.05,0 0,0
MULTIPLEXER  (via drill 1.2 pad 2.54)
  Top 2.54: D9.C 149.86,81.28 154.94,76.2 154.94,60.96 153.67,59.69 143.51,59.69 142.24,58.42 142.24,53.34 v163.83,31.75 172.72,22.86 201.93,22.86 203.2,21.59 203.2,13.97 207.01,10.16 232.41,10.16 234.95,12.7 234.95,27.94 240.03,33.02 240.03,44.45 237.49,46.99 237.49,50.8 246.38,59.69 250.19,59.69 251.46,60.96 251.46,76.2 246.38,81.28 D21.C | v50.8,67.31 26.67,67.31 v25.4,68.58
  Bottom 1.778: 100.33,215.9 102.87,213.36 SV2.26
  Bottom 2.54: D9.C 149.86,90.17 151.13,88.9 K9.1 | D21.C 246.38,90.17 247.65,88.9 K21.1 | K52.P1 50.47,66.98 v50.8,67.31 | v25.4,68.58 15.24,58.42 12.7,58.42 | 12.7,58.42 10.16,55.88 10.16,39.37 22.86,26.67 66.04,26.67 76.2,36.83 76.2,40.64 77.47,41.91 82.55,41.91 83.82,40.64 83.82,22.86 100.33,6.35 138.43,6.35 v163.83,31.75 | 12.7,58.42 12.7,200.66 31.75,219.71 78.74,219.71 82.55,215.9 100.33,215.9
N$1
  Bottom 2.54: D3.A 134.62,80.01 K3.2 129.54,74.93 123.19,74.93 114.3,83.82 D2.A 113.03,80.01 K2.2 107.95,74.93 102.87,74.93 99.06,78.74 99.06,97.79 90.17,106.68 86.69,106.68 K12.P1
N$3  (via drill 1.2 pad 2.54)
  Top 2.54: v146.05,92.71 v146.05,73.66
  Bottom 2.54: K11.S1 157.07,102.01 | 157.07,102.01 154.94,104.14 154.94,109.22 152.4,111.76 151.49,111.76 K11.O2 | K9.P2 150.8,68.91 v146.05,73.66 | 157.07,102.01 157.07,101.19 153.67,97.79 148.59,97.79 146.05,95.25 v146.05,92.71
N$4
  Bottom 2.54: K52.O1 45.49,67.08 50.8,72.39 50.8,73.46 K51.P2 50.47,75.87 52.07,77.47 57.15,77.47 60.96,81.28 60.96,87.35 K50.S2
N$5  (via drill 1.2 pad 2.54)
  Top 2.54: D16.C 227.33,13.97 226.06,15.24 226.06,24.13 234.95,33.02 v234.95,43.18 | v234.95,59.69 234.95,66.04 233.68,67.31 194.31,67.31 v187.96,73.66
  Bottom 2.54: D16.C 231.14,17.78 229.87,19.05 K16.1 | v234.95,43.18 237.49,45.72 237.49,57.15 v234.95,59.69 | K22.P1 183.21,68.91 v187.96,73.66
N$6  (via drill 1.2 pad 2.54)
  Top 2.54: v203.2,46.99 203.2,41.91 205.74,39.37 v210.82,39.37
  Bottom 2.54: K13.P2 207.21,39.37 v210.82,39.37 | v203.2,46.99 199.52,50.67 K14.S2 193.9,53.75 190.5,57.15 190.5,64.77 193.04,67.31 203.43,67.31 K14.O1
N$7  (via drill 1.2 pad 2.54)
  Top 2.54: v138.43,67.31 102.87,67.31 v95.25,74.93 | D4.C 130.81,13.97 129.54,15.24 129.54,24.13 138.43,33.02 v138.43,44.45
  Bottom 2.54: D4.C 134.62,17.78 133.35,19.05 K4.1 | v138.43,67.31 142.24,63.5 142.24,48.26 v138.43,44.45 | K10.P1 87.96,68.91 93.98,74.93 v95.25,74.93
N$8
  Bottom 2.54: K10.P2 78.54,68.58 77.47,68.58 74.93,66.04 74.93,58.42 77.47,55.88 88.9,55.88 91.44,58.42 91.44,67.31 95.25,71.12 130.81,71.12 138.43,78.74 138.43,85.09 135.89,87.63 D8.C 134.62,91.44 133.35,92.71 K8.1
N$9  (via drill 1.2 pad 2.54)
  Top 2.54: v116.84,49.53 v116.84,57.15
  Bottom 2.54: K2.P1 112.09,58.42 115.57,58.42 v116.84,57.15 | K4.S1 125.73,46.99 123.19,49.53 v116.84,49.53
N$10  (via drill 1.2 pad 2.54)
  Top 2.54: v107.95,46.99 107.95,40.64 109.22,39.37 v115.57,39.37
  Bottom 2.54: K2.O1 111.76,64.77 109.22,67.31 96.52,67.31 95.25,66.04 95.25,55.88 97.79,53.34 98.2,53.75 K2.S2 104.14,53.62 104.14,50.8 v107.95,46.99 | K1.P2 111.96,39.37 v115.57,39.37
N$11  (via drill 1.2 pad 2.54)
  Top 2.54: v107.95,120.65 107.95,115.57 110.49,113.03 v115.57,113.03
  Bottom 2.54: K6.O1 111.76,138.43 107.95,142.24 97.79,142.24 95.25,139.7 95.25,129.54 97.79,127 103.86,127 | 103.86,127 K6.S2 | 103.86,127 103.86,124.74 v107.95,120.65 | K5.P2 111.96,113.03 v115.57,113.03
N$12  (via drill 1.2 pad 2.54)
  Top 2.54: v99.06,39.37 99.06,46.99 95.25,50.8 95.25,59.69 v99.06,63.5
  Bottom 2.54: K3.S2 121.92,53.75 | 121.92,53.75 K2.S1 110.9,54.61 109.22,54.61 107.95,55.88 107.95,62.23 106.68,63.5 104.14,63.5 104.27,63.63 K2.O2 104.04,63.5 v99.06,63.5 | K3.O1 129.77,67.31 119.38,67.31 116.84,64.77 116.84,62.23 119.38,59.69 120.65,59.69 121.92,58.42 121.92,53.75 | K1.P1 103.81,39.37 v99.06,39.37
N$13  (via drill 1.2 pad 2.54)
  Top 2.54: v99.06,137.16 95.25,133.35 95.25,125.73 99.06,121.92 v99.06,113.03
  Bottom 2.54: K7.S2 121.92,127.41 | 121.92,127.41 K6.S1 110.9,128.27 109.22,128.27 107.95,129.54 107.95,135.89 106.45,137.39 K6.O2 99.29,137.39 v99.06,137.16 | K7.O1 133.12,137.39 129.54,140.97 119.38,140.97 116.84,138.43 116.84,135.89 119.38,133.35 120.65,133.35 121.92,132.08 121.92,127.41 | K5.P1 99.39,112.7 v99.06,113.03
N$14
  Bottom 2.54: K7.P2 129.54,128.73 129.54,109.22 131.04,107.72 K8.O2
N$15
  Bottom 2.54: K3.P2 129.54,55.07 129.54,35.56 131.04,34.06 K4.O2
N$16
  Bottom 2.54: K4.S2 138.43,49.25 138.43,55.88 135.56,58.75 K3.P1
N$17  (via drill 1.2 pad 2.54)
  Top 2.54: v120.65,34.29 120.65,40.64 110.49,50.8 101.6,50.8 99.06,53.34 v99.06,58.42
  Bottom 2.54: K4.O1 125.5,34.29 v120.65,34.29 | K2.P2 103.94,58.42 v99.06,58.42
N$18
  Bottom 2.54: K7.P1 135.56,132.41 138.43,129.54 138.43,122.91 K8.S2
N$19  (via drill 1.2 pad 2.54)
  Top 2.54: v99.06,132.08 99.06,127 101.6,124.46 110.49,124.46 120.65,114.3 v120.65,107.95
  Bottom 2.54: K6.P2 99.39,132.41 v99.06,132.08 | v120.65,107.95 120.88,107.72 K8.O1
N$20  (via drill 1.2 pad 2.54)
  Top 2.54: v116.84,130.81 v116.84,123.19
  Bottom 2.54: K6.P1 115.24,132.41 v116.84,130.81 | v116.84,123.19 123.19,123.19 125.73,120.65 K8.S1
N$21  (via drill 1.2 pad 2.54)
  Top 2.54: v194.31,39.37 194.31,48.26 190.5,52.07 190.5,59.69 v194.31,63.5
  Bottom 2.54: K15.S2 218.44,53.75 | 218.44,53.75 K14.S1 206.6,53.75 203.2,57.15 203.2,60.05 K14.O2 194.54,63.73 v194.31,63.5 | K13.P1 194.64,39.04 v194.31,39.37 | K15.O1 228.37,63.73 224.79,67.31 215.9,67.31 213.36,64.77 213.36,62.23 218.44,57.15 218.44,53.75
N$22
  Bottom 2.54: D7.A 134.62,153.67 K7.2 129.54,148.59 124.46,148.59 115.57,157.48 D6.A 113.03,153.67 K6.2 107.95,148.59 99.06,148.59 91.44,140.97 91.44,125.73 82.55,116.84 82.55,109.22 80.34,107.01 K12.P2
N$23
  Bottom 2.54: K15.P2 226.06,55.07 226.06,35.56 227.56,34.06 K16.O2
N$24
  Bottom 2.54: K15.P1 233.68,54.94 233.68,46.99 230.73,44.04 K16.S2
N$25  (via drill 1.2 pad 2.54)
  Top 2.54: v217.17,34.29 217.17,39.37 205.74,50.8 196.85,50.8 194.31,53.34 v194.31,58.42
  Bottom 2.54: K16.O1 222.25,34.29 v217.17,34.29 | K14.P2 199.52,58.55 199.39,58.42 v194.31,58.42
N$26  (via drill 1.2 pad 2.54)
  Top 2.54: v212.09,49.53 v212.09,57.15
  Bottom 2.54: K14.P1 208.61,57.15 v212.09,57.15 | K16.S1 222.25,45.72 218.44,49.53 v212.09,49.53
N$27
  Bottom 2.54: K22.P2 173.79,68.58 171.45,68.58 170.18,67.31 170.18,62.23 172.72,59.69 184.15,59.69 186.69,62.23 186.69,67.31 190.5,71.12 228.6,71.12 234.95,77.47 234.95,86.36 233.68,87.63 D20.C 231.14,91.44 229.87,92.71 K20.1
N$28  (via drill 1.2 pad 2.54)
  Top 2.54: v203.2,120.65 203.2,114.3 204.47,113.03 v210.82,113.03
  Bottom 2.54: K17.P2 207.21,113.03 v210.82,113.03 | v203.2,120.65 199.52,124.33 K18.S2 193.9,127.41 190.5,130.81 190.5,138.43 193.04,140.97 203.43,140.97 K18.O1
N$29  (via drill 1.2 pad 2.54)
  Top 2.54: v194.31,119.38 194.31,121.92 190.5,125.73 190.5,133.35 v194.31,137.16
  Bottom 2.54: v194.31,137.16 194.54,137.39 K18.O2 203.2,133.71 203.2,130.81 206.6,127.41 K18.S1 K19.S2 219.3,127.41 218.44,128.27 218.44,130.81 213.36,135.89 213.36,138.43 215.9,140.97 224.79,140.97 228.37,137.39 K19.O1 | v194.31,119.38 194.31,117.78 K17.P1
N$30
  Bottom 2.54: K19.P2 226.06,128.73 226.06,109.22 227.56,107.72 K20.O2
N$31
  Bottom 2.54: K19.P1 233.68,128.6 233.68,120.65 230.73,117.7 K20.S2
N$32  (via drill 1.2 pad 2.54)
  Top 2.54: v217.17,107.95 217.17,113.03 205.74,124.46 196.85,124.46 194.31,127 v194.31,132.08
  Bottom 2.54: K20.O1 217.4,107.72 v217.17,107.95 | K18.P2 194.64,132.41 v194.31,132.08
N$33  (via drill 1.2 pad 2.54)
  Top 2.54: v212.09,123.19 v212.09,130.81
  Bottom 2.54: K18.P1 208.61,130.81 v212.09,130.81 | K20.S1 222.25,119.38 218.44,123.19 v212.09,123.19
N$34
  Bottom 2.54: 208.28,80.01 D14.A 212.09,83.82 220.98,74.93 226.06,74.93 K15.2 231.14,80.01 D15.A | 208.28,80.01 K14.2 | 208.28,80.01 207.01,80.01 201.93,74.93 198.12,74.93 194.31,78.74 194.31,97.79 185.42,106.68 181.94,106.68 K24.P1
N$35
  Bottom 2.54: K18.2 208.28,153.67 D18.A 212.09,157.48 220.98,148.59 | D19.A 231.14,153.67 K19.2 226.06,148.59 220.98,148.59 | K24.P2 175.59,107.01 177.8,109.22 177.8,118.11 186.69,127 186.69,139.7 195.58,148.59 220.98,148.59
N$36  (via drill 1.2 pad 2.54)
  Top 2.54: v242.57,72.39 v242.57,95.25
  Bottom 2.54: K23.S1 253.59,102.01 253.37,102.23 | 253.37,102.23 251.46,104.14 251.46,109.22 248.92,111.76 248.01,111.76 K23.O2 | K21.P2 246.05,68.91 v242.57,72.39 | v242.57,95.25 245.11,97.79 248.92,97.79 253.37,102.23
N$71
  Bottom 2.54: K50.P1 50.47,101.27 53.34,104.14 58.42,104.14 59.69,102.87 59.69,99.06 68.58,90.17 68.58,78.74 63.5,73.66 63.5,46.99 68.58,41.91 68.58,39.37 64.77,35.56 55.6,35.56 K53.S2
N$72  (via drill 1.2 pad 2.54)
  Top 2.54: v40.64,49.53 40.64,57.15 41.91,58.42 53.34,58.42 55.88,60.96 v55.88,66.04 60.96,71.12 60.96,74.93 58.42,77.47 52.07,77.47 50.8,78.74 50.8,83.82 v53.34,86.36
  Bottom 2.54: K53.O2 K53.O1 45.49,43.41 45.72,43.18 45.72,44.45 v40.64,49.53 | K51.P1 50.47,83.49 v53.34,86.36 | K52.S1 55.47,65.63 v55.88,66.04
NEXT_BIT_1  (via drill 1.2 pad 2.54)
  Top 2.54: v158.75,144.78 v217.17,144.78
  Bottom 2.54: K9.P1 157.15,68.91 154.94,71.12 154.94,91.44 156.21,92.71 156.21,95.25 158.75,97.79 161.29,97.79 166.37,102.87 166.37,109.22 163.83,111.76 158.98,111.76 | 158.98,111.76 K11.O1 | 158.98,111.76 158.75,111.76 154.94,115.57 154.94,140.97 v158.75,144.78 | K23.S2 245.97,102.01 238.76,109.22 238.76,134.62 228.6,144.78 v217.17,144.78
NEXT_BIT_3
  Bottom 1.778: 118.11,204.47 SV2.34
  Bottom 2.54: K21.P1 253.67,68.91 251.46,71.12 251.46,93.98 255.27,97.79 257.81,97.79 260.35,100.33 260.35,102.87 262.89,105.41 262.89,110.49 261.62,111.76 255.5,111.76 K23.O1 255.04,111.99 251.46,115.57 251.46,148.59 207.01,193.04 134.62,193.04 133.35,194.31 133.35,203.2 128.27,208.28 123.19,208.28 119.38,204.47 118.11,204.47
NEXT_BIT_7  (via drill 1.2 pad 2.54)
  Top 2.54: v138.43,157.48 v138.43,177.8
  Bottom 1.778: 115.57,199.39 114.3,199.39 113.03,200.66 SV2.33
  Bottom 2.54: K11.S2 149.45,102.01 142.24,109.22 142.24,140.97 138.43,144.78 v138.43,157.48 | v138.43,177.8 135.89,177.8 129.54,184.15 129.54,201.93 127,204.47 124.46,204.47 119.38,199.39 115.57,199.39
NOT_A_0  (via drill 0.7 pad 1.78, 1.2 pad 2.54)
  Top 1.778: v6.35,199.39 50.8,199.39 v58.42,191.77
  Top 2.54: D5.A 96.52,93.98 92.71,93.98 91.44,92.71 91.44,88.9 86.36,83.82 86.36,80.01 91.44,74.93 91.44,49.53 v80.01,38.1
  Bottom 1.778: SV1.1 40.64,190.5 41.91,191.77 v58.42,191.77
  Bottom 2.54: D5.A 102.87,91.44 K5.2 | v6.35,199.39 6.35,38.1 21.59,22.86 68.58,22.86 80.01,34.29 v80.01,38.1
NOT_A_1  (via drill 0.7 pad 1.78)
  Top 1.778: 27.94,181.61 40.64,194.31 v48.26,194.31
  Top 2.54: D1.A 97.79,13.97 85.09,26.67 22.86,26.67 17.78,31.75 17.78,41.91 21.59,45.72 21.59,62.23 17.78,66.04 17.78,114.3 21.59,118.11 21.59,121.92 27.94,128.27 27.94,181.61
  Bottom 1.778: SV1.3 39.37,186.69 38.1,187.96 38.1,191.77 40.64,194.31 v48.26,194.31
  Bottom 2.54: D1.A 102.87,17.78 K1.2
NOT_A_2  (via drill 0.7 pad 1.78, 1.2 pad 2.54)
  Top 2.54: D17.A 187.96,87.63 177.8,77.47 177.8,40.64 v186.69,30.48 | v147.32,198.12 138.43,198.12 135.89,195.58 96.52,195.58 93.98,193.04 62.23,193.04 v60.96,194.31
  Bottom 1.778: SV1.5 38.1,184.15 35.56,186.69 35.56,193.04 39.37,196.85 58.42,196.85 v60.96,194.31
  Bottom 2.54: D17.A 198.12,91.44 K17.2 | v186.69,30.48 186.69,13.97 190.5,10.16 232.41,10.16 234.95,12.7 234.95,27.94 262.89,55.88 262.89,73.66 255.27,81.28 255.27,82.55 260.35,87.63 260.35,93.98 266.7,100.33 266.7,111.76 261.62,116.84 261.62,132.08 255.27,138.43 255.27,162.56 219.71,198.12 v147.32,198.12
NOT_A_3  (via drill 0.7 pad 1.78)
  Top 1.778: 24.13,185.42 v33.02,194.31
  Top 2.54: D13.A 175.26,13.97 162.56,26.67 142.24,26.67 139.7,24.13 139.7,12.7 137.16,10.16 96.52,10.16 83.82,22.86 21.59,22.86 13.97,30.48 13.97,43.18 17.78,46.99 17.78,60.96 13.97,64.77 13.97,115.57 17.78,119.38 17.78,123.19 24.13,129.54 24.13,185.42
  Bottom 1.778: SV1.7 36.83,181.61 33.02,185.42 v33.02,194.31
  Bottom 2.54: D13.A 198.12,17.78 K13.2
NOT_A_4
  Bottom 1.778: SV1.9 35.56,179.07 30.48,184.15 30.48,195.58 36.83,201.93 67.31,201.93 69.85,204.47 SV2.2
NOT_A_5
  Bottom 1.778: SV1.11 34.29,176.53 27.94,182.88 27.94,196.85 35.56,204.47 66.04,204.47 68.58,207.01 73.66,207.01 74.93,205.74 SV2.4
NOT_A_6
  Bottom 1.778: SV1.13 33.02,173.99 25.4,181.61 25.4,198.12 34.29,207.01 64.77,207.01 67.31,209.55 74.93,209.55 77.47,207.01 SV2.6
NOT_A_7
  Bottom 1.778: SV1.15 31.75,171.45 22.86,180.34 22.86,199.39 33.02,209.55 63.5,209.55 66.04,212.09 76.2,212.09 80.01,208.28 SV2.8
NOT_B_0  (via drill 1.2 pad 2.54)
  Top 2.54: v66.04,111.76 v73.66,111.76
  Bottom 1.778: SV1.19 31.75,166.37 22.86,157.48 22.86,138.43 33.02,128.27 53.34,128.27 66.04,115.57 v66.04,111.76
  Bottom 2.54: K12.O2 73.89,111.99 v73.66,111.76
NOT_B_1  (via drill 1.2 pad 2.54)
  Top 2.54: v66.04,120.65 71.12,115.57 88.9,115.57 v91.44,113.03
  Bottom 1.778: SV1.21 33.02,163.83 25.4,156.21 25.4,139.7 34.29,130.81 55.88,130.81 v66.04,120.65
  Bottom 2.54: K12.O1 90.4,111.99 v91.44,113.03
NOT_B_2
  Bottom 1.778: SV1.23 34.29,161.29 27.94,154.94 27.94,140.97 35.56,133.35 73.66,133.35 76.2,135.89
  Bottom 2.54: K24.O2 174.12,121.79 168.91,127 168.91,148.59 151.13,166.37 133.35,166.37 128.27,161.29 101.6,161.29 99.06,158.75 99.06,153.67 81.28,135.89 76.2,135.89
NOT_B_3  (via drill 1.2 pad 2.54)
  Top 2.54: v154.94,170.18 154.94,124.46 156.21,123.19 172.72,123.19 185.42,110.49 v186.69,110.49
  Bottom 1.778: SV1.25 35.56,158.75 30.48,153.67 30.48,142.24 36.83,135.89 71.12,135.89 74.93,139.7
  Bottom 2.54: 74.93,139.7 78.74,139.7 95.25,156.21 95.25,161.29 99.06,165.1 127,165.1 132.08,170.18 v154.94,170.18 | K24.O1 185.19,111.99 v186.69,110.49
NOT_B_4
  Bottom 1.778: SV1.27 36.83,156.21 33.02,152.4 33.02,143.51 38.1,138.43 53.34,138.43 102.87,187.96 SV2.25
NOT_B_5
  Bottom 1.778: SV1.29 38.1,153.67 35.56,151.13 35.56,144.78 39.37,140.97 52.07,140.97 100.33,189.23 SV2.23
NOT_B_6
  Bottom 1.778: SV1.31 39.37,151.13 38.1,149.86 38.1,146.05 40.64,143.51 50.8,143.51 97.79,190.5 SV2.21
NOT_B_7
  Bottom 1.778: SV1.33 40.64,147.32 41.91,146.05 49.53,146.05 95.25,191.77 SV2.19
NOT_I_0  (via drill 0.7 pad 1.78, 1.2 pad 2.54)
  Top 1.778: v26.67,106.68 31.75,106.68 36.83,111.76 36.83,129.54 53.34,146.05 v53.34,160.02
  Bottom 1.778: SV1.24 52.07,161.29 v53.34,160.02
  Bottom 2.54: D51.A 29.21,82.55 | 29.21,82.55 K51.2 | 29.21,82.55 21.59,90.17 21.59,104.14 24.13,106.68 v26.67,106.68
NOT_I_1  (via drill 0.7 pad 1.78)
  Top 1.778: D50.A 21.59,105.41 21.59,111.76 25.4,115.57 31.75,115.57 34.29,118.11 34.29,130.81 50.8,147.32 v50.8,158.75
  Top 2.54: D50.A 25.4,96.52 21.59,92.71 21.59,67.31 D52.A
  Bottom 1.778: SV1.26 v50.8,158.75
  Bottom 2.54: D50.A 29.21,101.6 K50.2 | D52.A 29.21,63.5 K52.2
NOT_I_2  (via drill 0.7 pad 1.78)
  Top 1.778: v48.26,156.21 48.26,148.59 31.75,132.08 31.75,127 D49.A
  Bottom 1.778: SV1.28 v48.26,156.21
  Bottom 2.54: D49.A 29.21,120.65 K49.2
RESULT_0  (via drill 0.7 pad 1.78, 1.2 pad 2.54)
  Top 1.778: v55.88,189.23 128.27,189.23 130.81,191.77 139.7,191.77 142.24,189.23 v142.24,185.42
  Top 2.54: v146.05,157.48 v146.05,177.8
  Bottom 1.778: SV1.2 v55.88,189.23
  Bottom 2.54: K11.P2 149.53,107.01 146.05,110.49 v146.05,157.48 | v146.05,177.8 146.05,181.61 v142.24,185.42
RESULT_1  (via drill 0.7 pad 1.78, 1.2 pad 2.54)
  Top 1.778: v53.34,186.69 129.54,186.69 132.08,189.23 135.89,189.23 137.16,187.96 v137.16,185.42
  Top 2.54: v162.56,106.68 162.56,116.84 160.02,119.38 153.67,119.38 146.05,127 146.05,142.24 142.24,146.05 v142.24,177.8
  Bottom 1.778: SV1.4 v53.34,186.69
  Bottom 2.54: K11.P1 159.69,107.01 160.02,106.68 v162.56,106.68 | v142.24,177.8 142.24,180.34 v137.16,185.42
RESULT_2  (via drill 0.7 pad 1.78, 1.2 pad 2.54)
  Top 1.778: v133.35,185.42 132.08,184.15 v50.8,184.15
  Bottom 1.778: SV1.6 v50.8,184.15
  Bottom 2.54: K23.P2 246.05,107.01 242.57,110.49 242.57,151.13 204.47,189.23 134.62,189.23 133.35,187.96 v133.35,185.42
RESULT_3  (via drill 0.7 pad 1.78, 1.2 pad 2.54)
  Top 1.778: v48.26,181.61 138.43,181.61
  Top 2.54: v259.08,107.95 259.08,114.3 251.46,121.92 251.46,152.4 222.25,181.61 138.43,181.61
  Bottom 1.778: SV1.8 v48.26,181.61
  Bottom 2.54: K23.P1 258.14,107.01 v259.08,107.95
RESULT_4
  Bottom 1.778: SV1.10 49.53,179.07 SV2.1
RESULT_5
  Bottom 1.778: SV1.12 50.8,176.53 74.93,200.66 SV2.3
RESULT_6
  Bottom 1.778: SV1.14 52.07,173.99 77.47,199.39 SV2.5
RESULT_7
  Bottom 1.778: SV1.16 53.34,171.45 80.01,198.12 SV2.7
SHIFTER  (via drill 1.2 pad 2.54)
  Top 2.54: D11.C v149.86,173.99 223.52,173.99 246.38,151.13 D23.C | v49.53,87.63 44.45,87.63 34.29,77.47 v25.4,77.47 | v96.52,212.09 114.3,212.09 v125.73,200.66
  Bottom 1.778: v96.52,212.09 97.79,210.82 SV2.22
  Bottom 2.54: D11.C 149.86,128.27 151.13,127 K11.1 | D23.C 246.38,128.27 247.65,127 K23.1 | K50.P2 50.47,88.57 v49.53,87.63 | v25.4,77.47 24.13,77.47 17.78,83.82 17.78,127 16.51,128.27 16.51,133.35 17.78,134.62 17.78,199.39 34.29,215.9 77.47,215.9 81.28,212.09 v96.52,212.09 | v125.73,200.66 125.73,182.88 134.62,173.99 v149.86,173.99
SUM_0  (via drill 1.2 pad 2.54)
  Top 2.54: v120.65,100.33 v140.97,100.33
  Bottom 2.54: K8.P1 124.79,111.76 119.38,111.76 116.84,109.22 116.84,106.68 120.65,102.87 v120.65,100.33 | v140.97,100.33 140.97,95.25 142.24,93.98 142.24,91.44 146.05,87.63 146.05,79.1 K9.O2
SUM_1
  Bottom 2.54: K4.P1 124.79,38.1 119.38,38.1 116.84,35.56 116.84,33.02 119.38,30.48 135.89,30.48 149.86,44.45 149.86,54.61 151.13,55.88 156.21,55.88 162.56,62.23 162.56,71.12 159.79,73.89 K9.O1
SUM_2  (via drill 1.2 pad 2.54)
  Top 2.54: v217.17,100.33 226.06,100.33 229.87,104.14 v237.49,104.14
  Bottom 2.54: K20.P1 216.84,112.7 213.36,109.22 213.36,106.68 217.17,102.87 v217.17,100.33 | K21.O2 242.57,79.1 242.57,88.9 238.76,92.71 238.76,95.25 237.49,96.52 v237.49,104.14
SUM_3
  Bottom 2.54: K16.P1 216.84,39.04 213.36,35.56 213.36,33.02 217.17,29.21 231.14,29.21 245.11,43.18 245.11,54.61 246.38,55.88 252.73,55.88 259.08,62.23 259.08,71.12 256.54,73.66 255.5,73.66 K21.O1

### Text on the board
tRestrict: A Relay Based Processor / ALU Bits 0 Thru 3 / Topside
